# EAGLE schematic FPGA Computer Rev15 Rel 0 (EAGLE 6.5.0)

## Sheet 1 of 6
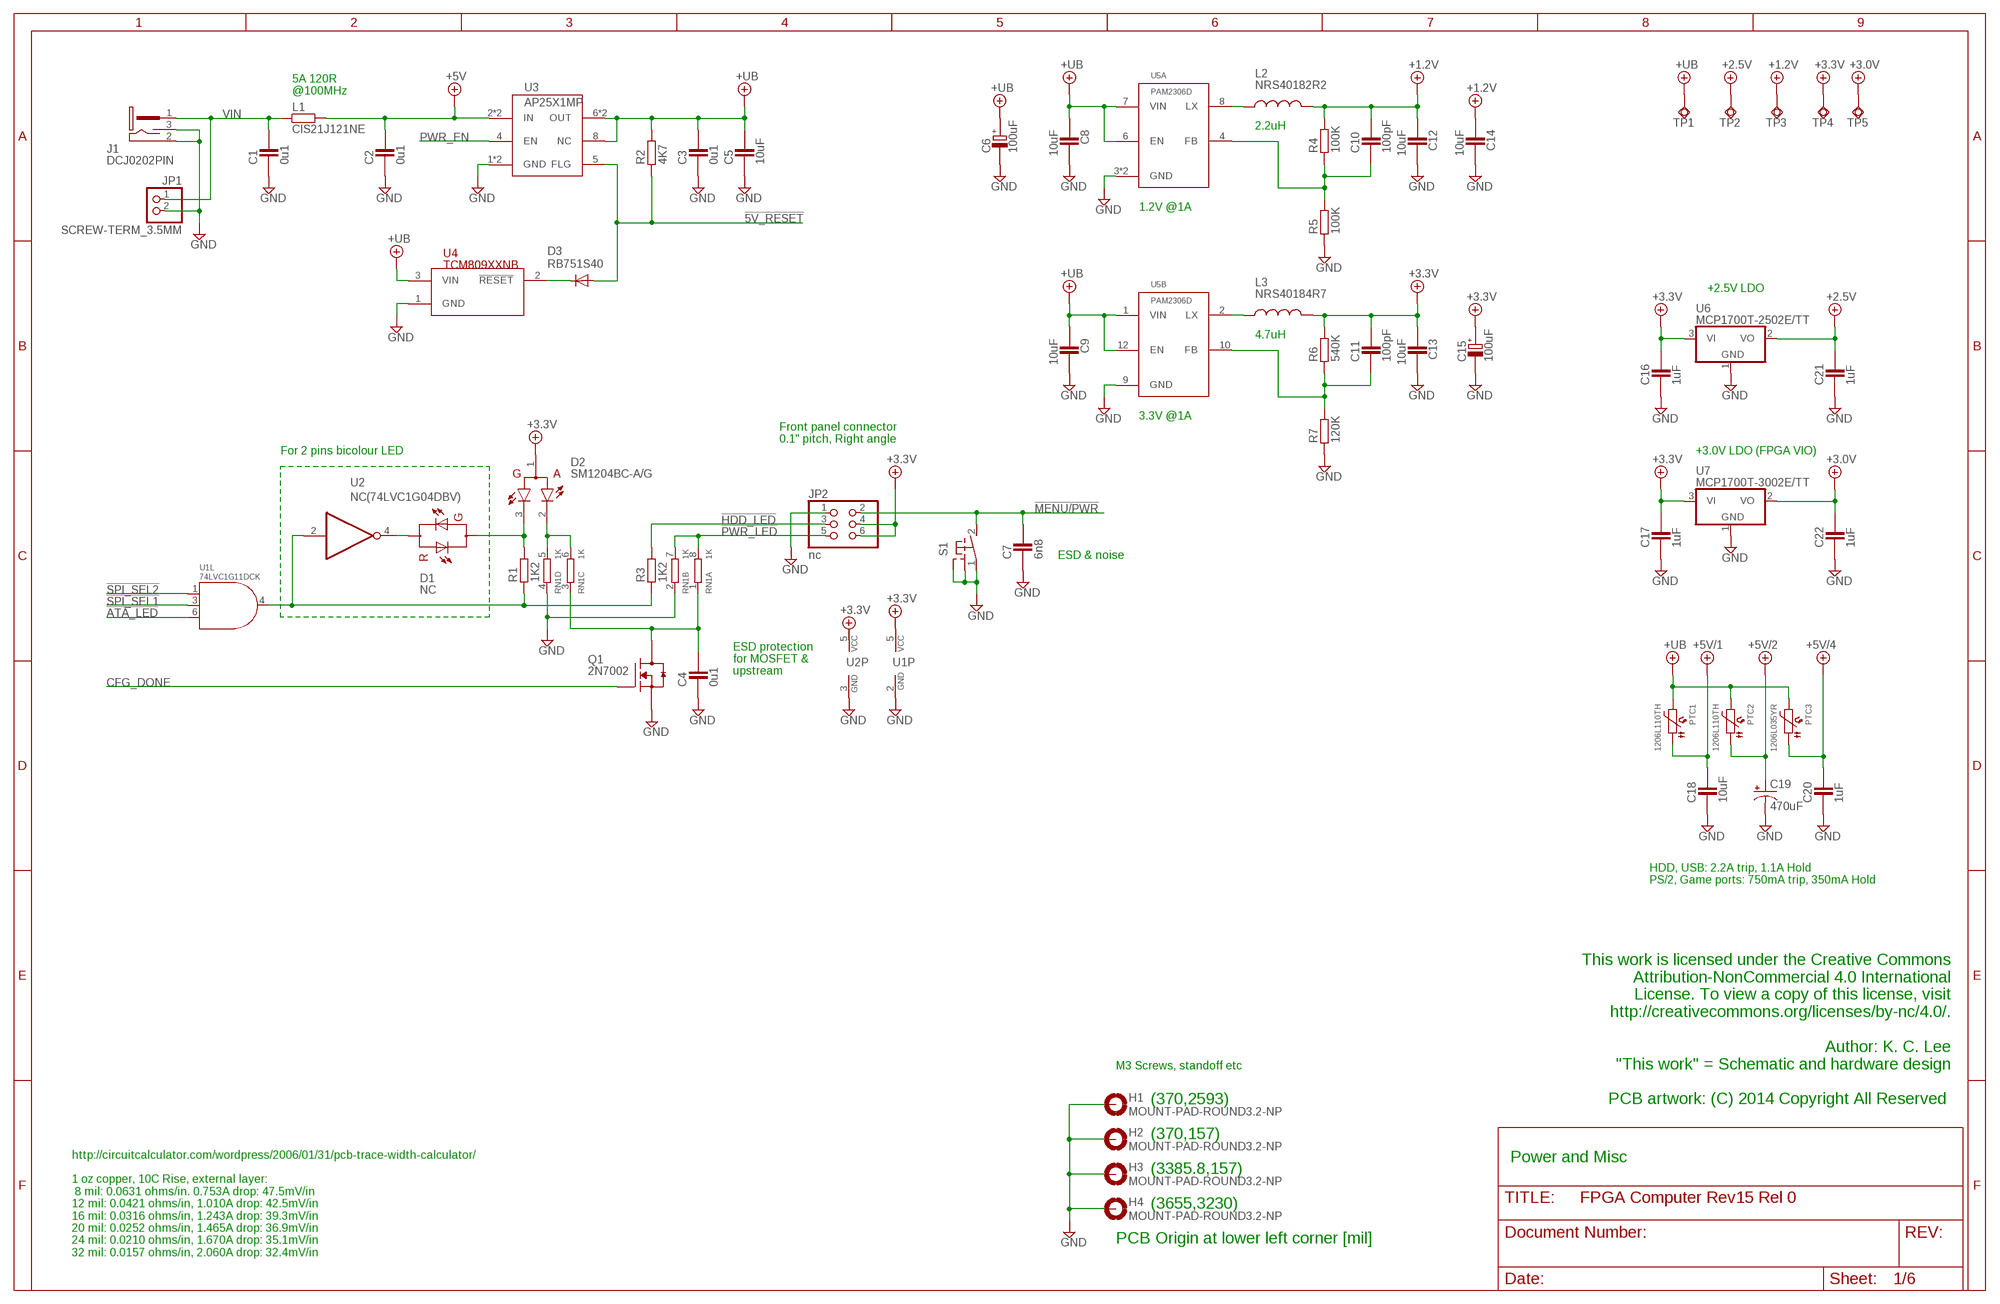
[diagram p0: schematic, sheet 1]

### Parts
C1  0u1  CAPACITOR_0603  [CAPC1608X92N]
C2  0u1  CAPACITOR_0603  [CAPC1608X92N]
C3  0u1  CAPACITOR_0603  [CAPC1608X92N]
C4  0u1  CAPACITOR_0603  [CAPC1608X92N]
C5  10uF  CAPACITOR_0805N  [CAP2012X70N]
C6  100uF  POLARISED_D_CASE  [CAPMP7343X310N]
C7  6n8  CAPACITOR_0603  [CAPC1608X92N]
C8  10uF  CAPACITOR_0805N  [CAP2012X70N]
C9  10uF  CAPACITOR_0805N  [CAP2012X70N]
C10  100pF  CAPACITOR_0603  [CAPC1608X92N]
C11  100pF  CAPACITOR_0603  [CAPC1608X92N]
C12  10uF  CAPACITOR_0805N  [CAP2012X70N]
C13  10uF  CAPACITOR_0805N  [CAP2012X70N]
C14  10uF  CAPACITOR_0805N  [CAP2012X70N]
C15  100uF  POLARISED_D_CASE  [CAPMP7343X310N]
C16  1uF  CAPACITOR_0603  [CAPC1608X92N]
C17  1uF  CAPACITOR_0603  [CAPC1608X92N]
C18  10uF  CAPACITOR_0805N  [CAP2012X70N]
C19  470uF  CAP_POL  [E2,5-6E]
C20  1uF  CAPACITOR_0603  [CAPC1608X92N]
C21  1uF  CAPACITOR_0603  [CAPC1608X92N]
C22  1uF  CAPACITOR_0603  [CAPC1608X92N]
D1  NC  DUAL-LED3MM  [LED3MM]
D2  SM1204BC-A/G  1204-SIDE-DUAL-AG  [LED_1204]
D3  RB751S40  DIODE-SOD523  [SOD523]
H1  MOUNT-PAD-ROUND3.2-NP  [3.2-PAD-NP]
H2  MOUNT-PAD-ROUND3.2-NP  [3.2-PAD-NP]
H3  MOUNT-PAD-ROUND3.2-NP  [3.2-PAD-NP]
H4  MOUNT-PAD-ROUND3.2-NP  [3.2-PAD-NP]
J1  DCJ0202PIN  [PJ-102A]
JP1  SCREW-TERM_3.5MM  [SCREWTERMINAL-3.5MM-2]
JP2  nc  PINHD-2X3_2.54-90°  [2X03-90]
L1  CIS21J121NE  RESISTOR_0805  [RESC2012X70N]
L2  NRS40182R2  NRS4018  [NR4018]
L3  NRS40184R7  NRS4018  [NR4018]
PTC1  1206L110TH  PTC1206  [1206]
PTC2  1206L110TH  PTC1206  [1206]
PTC3  1206L035YR  PTC1206  [1206]
Q1  2N7002  MOSFET-NCH_SOT-23  [SOT95P280X135-3N]
R1  1K2  RESISTOR_0603  [RESC1608X55N]
R2  4K7  RESISTOR_0603  [RESC1608X55N]
R3  1K2  RESISTOR_0603  [RESC1608X55N]
R4  100K  RESISTOR_0603  [RESC1608X55N]
R5  100K  RESISTOR_0603  [RESC1608X55N]
R6  540K  RESISTOR_0603  [RESC1608X55N]
R7  120K  RESISTOR_0603  [RESC1608X55N]
RN1  1K  4R-NCAT16  [CAT16]
S1  MOM_SW-RTPTS635V  [PTS635V]
TP1  TPSQTP07R  [TP07R]
TP2  TPSQTP07R  [TP07R]
TP3  TPSQTP07R  [TP07R]
TP4  TPSQTP07R  [TP07R]
TP5  TPSQTP07R  [TP07R]
U1  74LVC1G11DCK  [SC70-6]
U2  NC(74LVC1G04DBV)  74LVC1G04DBV  [SOT23-5]
U3  AP25X1MP  [MSOP8-PAD]
U4  TCM809XXNB  [SOT95P280X135-3N]
U5  PAM2306D  [PAM2306D]
U6  MCP1700T-2502E/TT  MCP1700/TT  [SOT95P280X135-3N]
U7  MCP1700T-3002E/TT  MCP1700/TT  [SOT95P280X135-3N]

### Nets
!5V_RESET: D3.A R2.1 U3.5(FLG) ; also sheet 3
!5V_RESET1: R1.1 R3.1 U1.4(L:Y) U2.2(I)
!ATA_LED: U1.6(L:C) ; also sheet 3
!HDD_LED: JP2.3 R3.2
!MENU/PWR: C7.2 JP2.2 S1.2(S) ; also sheet 4
!PWR_LED: JP2.5 RN1.7 RN1.8
!SPI_SEL1: U1.3(L:B) ; also sheet 2,4
!SPI_SEL2: U1.1(L:A) ; also sheet 2,4
+1.2V: C10.2 C12.1 C14.1 L2.2 R4.2 TP3.TP ; also sheet 5,6
+2.5V: C21.2 TP2.TP U6.2(VO) ; also sheet 5,6
+3.0V: C22.2 TP5.TP U7.2(VO) ; also sheet 5,6
+3.3V: C11.2 C13.1 C15.+ C16.2 C17.2 D2.1(A) JP2.4 JP2.6 L3.2 R6.2 TP4.TP U1.5(P:VCC) U2.5(VCC) U6.3(VI) U7.3(VI) ; also sheet 2,3,5
+5V: C2.2 L1.2 U3.2(IN) U3.3(IN) ; also sheet 4
+5V/1: C18.2 PTC1.1 ; also sheet 3
+5V/2: C19.+ PTC2.1 ; also sheet 4
+5V/4: C20.2 PTC3.1 ; also sheet 2
+UB: C3.2 C5.2 C6.+ C8.1 C9.1 PTC1.2 PTC2.2 PTC3.2 R2.2 TP1.TP U3.6(OUT) U3.7(OUT) U3.8(NC) U4.3(VIN) U5.1(B:VIN) U5.6(A:EN) U5.7(A:VIN) U5.12(B:EN) ; also sheet 2,5,6
CFG_DONE: Q1.1(G) ; also sheet 4,5
GND: C1.1 C2.1 C3.1 C4.1 C5.1 C6.- C7.1 C8.2 C9.2 C12.2 C13.2 C14.2 C15.- C16.1 C17.1 C18.1 C19.- C20.1 C21.1 C22.1 H1.H@1(MOUNT) H1.H@2(MOUNT) H1.H@3(MOUNT) H1.H@4(MOUNT) H1.H@5(MOUNT) H1.H@6(MOUNT) H1.H@7(MOUNT) H1.H@8(MOUNT) H2.H@1(MOUNT) H2.H@2(MOUNT) H2.H@3(MOUNT) H2.H@4(MOUNT) H2.H@5(MOUNT) H2.H@6(MOUNT) H2.H@7(MOUNT) H2.H@8(MOUNT) H3.H@1(MOUNT) H3.H@2(MOUNT) H3.H@3(MOUNT) H3.H@4(MOUNT) H3.H@5(MOUNT) H3.H@6(MOUNT) H3.H@7(MOUNT) H3.H@8(MOUNT) H4.H@1(MOUNT) H4.H@2(MOUNT) H4.H@3(MOUNT) H4.H@4(MOUNT) H4.H@5(MOUNT) H4.H@6(MOUNT) H4.H@7(MOUNT) H4.H@8(MOUNT) J1.2 J1.3 JP1.2 JP2.1 Q1.2(S) R5.1 R7.1 RN1.2 RN1.4 S1.1(P) S1.3(SHD) S1.4(SHD) U1.2(P:GND) U2.3(GND) U3.1(GND) U3.PAD(GND) U4.1(GND) U5.3(A:GND) U5.9(B:GND) U5.PAD(A:GND) U6.1(GND) U7.1(GND) ; also sheet 2,3,4,5,6
N$5: D3.C U4.2(!RESET)
N$25: D2.2(C2) RN1.5 RN1.6
N$60: C4.2 Q1.3(D) RN1.1 RN1.3
N$65: D1.A D2.3(C1) R1.2
N$84: C10.1 R4.1 R5.2 U5.4(A:FB)
N$85: L2.1 U5.8(A:LX)
N$87: C11.1 R6.1 R7.2 U5.10(B:FB)
N$88: L3.1 U5.2(B:LX)
N$98: D1.K(C) U2.4(O)
PWR_EN: U3.4(EN) ; also sheet 4
VIN: C1.2 J1.1 JP1.1 L1.1

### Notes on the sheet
- 5A 120R
  @100MHz
- 2.2uH
- 1.2V @1A
- +2.5V LDO
- 4.7uH
- 3.3V @1A
- Front panel connector
  0.1" pitch, Right angle
- For 2 pins bicolour LED | +3.0V LDO (FPGA VIO)
- ESD & noise
- ESD protection
  for MOSFET &
  upstream
- HDD, USB: 2.2A trip, 1.1A Hold
  PS/2, Game ports: 750mA trip, 350mA Hold
- M3 Screws, standoff etc
- (370,2593)
- This work is licensed under the Creative Commons
  Attribution-NonCommercial 4.0 International
  License. To view a copy of this license, visit
  http://creativecommons.org/licenses/by-nc/4.0/.
  
  Author: K. C. Lee
  "This work" = Schematic and hardware design
  
  PCB artwork: (C) 2014 Copyright All Reserved
- (370,157)
- http://circuitcalculator.com/wordpress/2006/01/31/pcb-trace-width-calculator/
  
  1 oz copper, 10C Rise, external layer:
   8 mil: 0.0631 ohms/in. 0.753A drop: 47.5mV/in
  12 mil: 0.0421 ohms/in, 1.010A drop: 42.5mV/in
  16 mil: 0.0316 ohms/in, 1.243A drop: 39.3mV/in
  20 mil: 0.0252 ohms/in, 1.465A drop: 36.9mV/in
  24 mil: 0.0210 ohms/in, 1.670A drop: 35.1mV/in
  32 mil: 0.0157 ohms/in, 2.060A drop: 32.4mV/in
- Power and Misc
- (3385.8,157)
- (3655,3230)
- PCB Origin at lower left corner [mil]

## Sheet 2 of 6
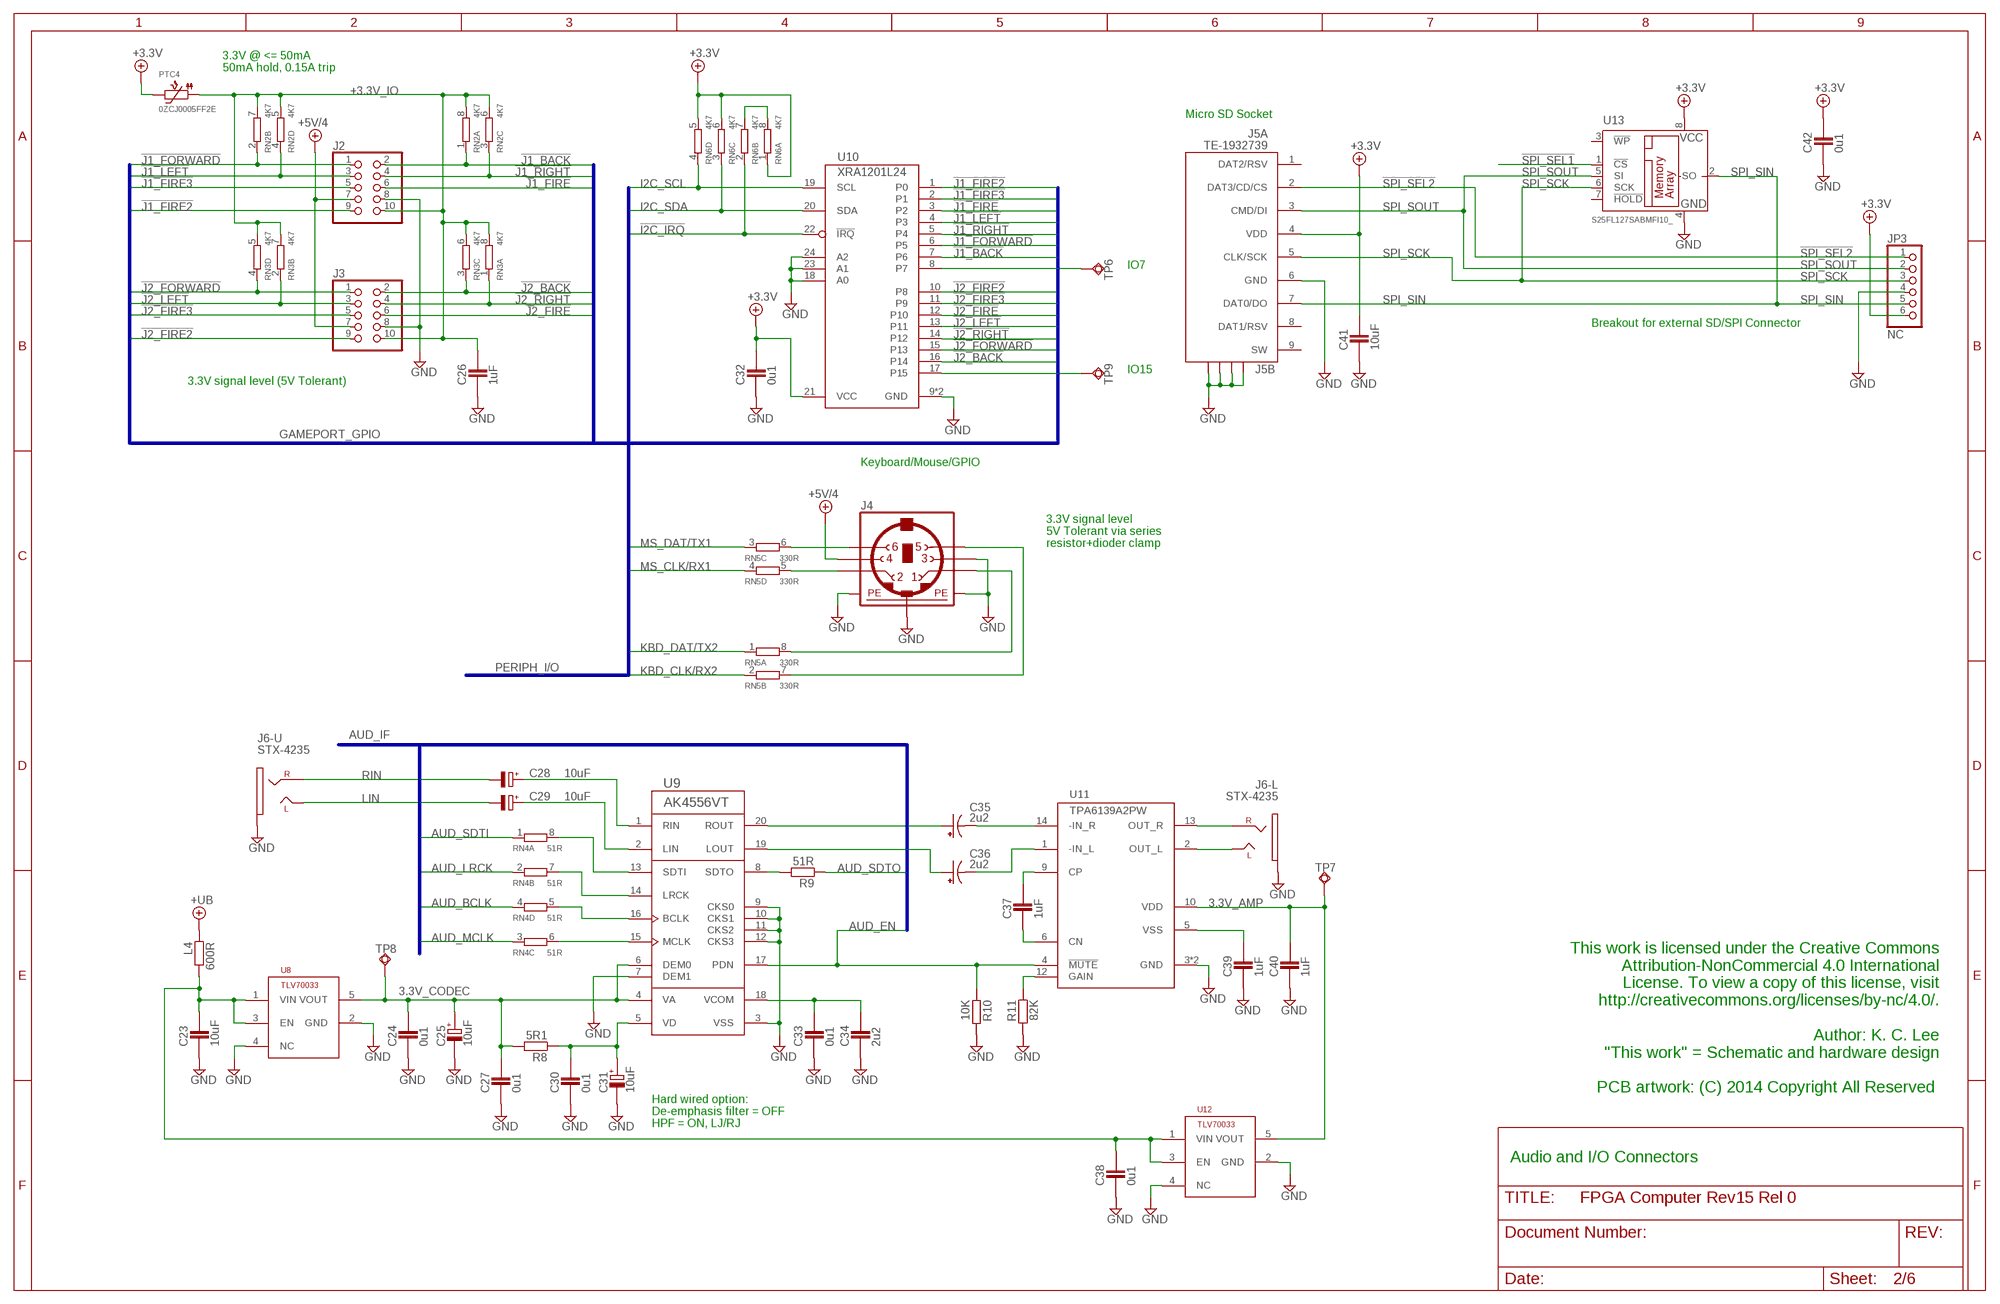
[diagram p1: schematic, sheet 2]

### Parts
C23  10uF  CAPACITOR_0805N  [CAP2012X70N]
C24  0u1  CAPACITOR_0603  [CAPC1608X92N]
C25  10uF  POLARISED_B_CASE  [CAPMP3528X210N]
C26  1uF  CAPACITOR_0603  [CAPC1608X92N]
C27  0u1  CAPACITOR_0603  [CAPC1608X92N]
C28  10uF  CPOL-EUE2-5  [E2-5]
C29  10uF  CPOL-EUE2-5  [E2-5]
C30  0u1  CAPACITOR_0603  [CAPC1608X92N]
C31  10uF  POLARISED_B_CASE  [CAPMP3528X210N]
C32  0u1  CAPACITOR_0603  [CAPC1608X92N]
C33  0u1  CAPACITOR_0603  [CAPC1608X92N]
C34  2u2  CAPACITOR_0603  [CAPC1608X92N]
C35  2u2  C-PR-1,0X3  [E1,0-3]
C36  2u2  C-PR-1,0X3  [E1,0-3]
C37  1uF  CAPACITOR_0603  [CAPC1608X92N]
C38  0u1  CAPACITOR_0603  [CAPC1608X92N]
C39  1uF  CAPACITOR_0603  [CAPC1608X92N]
C40  1uF  CAPACITOR_0603  [CAPC1608X92N]
C41  10uF  CAPACITOR_0805N  [CAP2012X70N]
C42  0u1  CAPACITOR_0603  [CAPC1608X92N]
J2  PINHD-2X5_2.54-W/PLUG  [2X05-W_PLUG]
J3  PINHD-2X5_2.54-W/PLUG  [2X05-W_PLUG]
J4  MINI_DIN_6  [M_DIN6]
J5  TE-1932739  [TE-1932739]
J6  STX-4235  [STX-4235-3]
JP3  NC  PINHD-1X6_2.00  [1X06M]
L4  600R  RESISTOR_0603  [RESC1608X55N]
PTC4  0ZCJ0005FF2E  PTC1206  [1206]
R8  5R1  RESISTOR_0603  [RESC1608X55N]
R9  51R  RESISTOR_0603  [RESC1608X55N]
R10  10K  RESISTOR_0603  [RESC1608X55N]
R11  82K  RESISTOR_0603  [RESC1608X55N]
RN2  4K7  4R-NCAT16  [CAT16]
RN3  4K7  4R-NCAT16  [CAT16]
RN4  51R  4R-NCAT16  [CAT16]
RN5  330R  4R-NCAT16  [CAT16]
RN6  4K7  4R-NCAT16  [CAT16]
TP6  TPSQTP07R  [TP07R]
TP7  TPSQTP07R  [TP07R]
TP8  TPSQTP07R  [TP07R]
TP9  TPSQTP07R  [TP07R]
U8  TLV70033  LDO-5  [SOT23-5]
U9  AK4556VT  [TSSOP20]
U10  XRA1201L24  [S-PQFP-N24-PAD]
U11  TPA6139A2PW  [TSSOP14]
U12  TLV70033  LDO-5  [SOT23-5]
U13  S25FL127SABMFI10_  25LC080SN  [SO-08]

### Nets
3.3V_AMP: C40.2 TP7.TP U11.10(VDD) U12.5(VOUT)
3.3V_CODEC: C24.2 C25.+ C27.2 R8.2 TP8.TP U8.5(VOUT) U9.4(VA) U9.6(DEM0)
!I2C_IRQ: RN6.2 U10.22(!IRQ) ; also sheet 4,6
!J1_BACK: J2.2 RN2.1 U10.7(P6)
!J1_FIRE: J2.6 U10.3(P2)
!J1_FIRE2: J2.9 U10.1(P0)
!J1_FIRE3: J2.5 U10.2(P1)
!J1_FORWARD: J2.1 RN2.2 U10.6(P5)
!J1_LEFT: J2.3 RN2.4 U10.4(P3)
!J1_RIGHT: J2.4 RN2.3 U10.5(P4)
!J2_BACK: J3.2 RN3.3 U10.16(P14)
!J2_FIRE: J3.6 U10.12(P10)
!J2_FIRE2: J3.9 U10.10(P8)
!J2_FIRE3: J3.5 U10.11(P9)
!J2_FORWARD: J3.1 RN3.4 U10.15(P13)
!J2_LEFT: J3.3 RN3.2 U10.13(P11)
!J2_RIGHT: J3.4 RN3.1 U10.14(P12)
!SPI_SEL1: U13.1(!CS) ; also sheet 1,4
!SPI_SEL2: J5.2(A:DAT3/CD/CS) JP3.1 ; also sheet 1,4
+3.3V: C32.2 C41.2 C42.2 J5.4(A:VDD) JP3.6 PTC4.2 RN6.1 RN6.5 RN6.6 U10.21(VCC) U13.8(VCC) ; also sheet 1,3,5
+3.3V_IO: C26.2 J2.10 J3.10 PTC4.1 RN2.5 RN2.6 RN2.7 RN2.8 RN3.5 RN3.6 RN3.7 RN3.8
+5V/4: J2.7 J3.7 J4.4 ; also sheet 1
+UB: L4.1 ; also sheet 1,5,6
AUD_BCLK: RN4.4 ; also sheet 5
AUD_EN: R10.1 U9.17(PDN) U11.4(!MUTE) ; also sheet 6
AUD_LRCK: RN4.2 ; also sheet 5
AUD_MCLK: RN4.3 ; also sheet 5
AUD_SDTI: RN4.1 ; also sheet 5
AUD_SDTO: R9.1 ; also sheet 5
GND: C23.1 C24.1 C25.- C26.1 C27.1 C30.1 C31.- C32.1 C33.1 C34.1 C38.1 C39.1 C40.1 C41.1 C42.1 J2.8 J3.8 J4.3 J4.SH1(PE1) J4.SH2(PE2) J4.SH3(PE3) J5.6(A:GND) J5.G1(B:S1) J5.G2(B:S2) J5.G3(B:S3) J5.G4(B:S4) J6.5L J6.5U JP3.4 R10.2 R11.2 U8.2(GND) U8.4(NC) U9.3(VSS) U9.7(DEM1) U9.9(CKS0) U9.10(CKS1) U9.11(CKS2) U9.12(CKS3) U10.9(GND) U10.18(A0) U10.23(A1) U10.24(A2) U10.PAD(GND) U11.3(GND) U11.11(GND) U12.2(GND) U12.4(NC) U13.4(GND) ; also sheet 1,3,4,5,6
I2C_SCL: RN6.4 U10.19(SCL) ; also sheet 4,6
I2C_SDA: RN6.3 U10.20(SDA) ; also sheet 4,6
KBD_CLK/RX2: RN5.2 ; also sheet 4
KBD_DAT/TX2: RN5.1 ; also sheet 4
LIN: C29.- J6.4U
MS_CLK/RX1: RN5.4 ; also sheet 4
MS_DAT/TX1: RN5.3 ; also sheet 4
N$1: J4.6 RN5.6
N$9: C23.2 C38.2 L4.2 U8.1(VIN) U8.3(EN) U12.1(VIN) U12.3(EN)
N$12: C36.- U11.1(-IN_L)
N$15: RN6.7 RN6.8
N$17: J4.1 RN5.8
N$19: J4.5 RN5.7
N$20: R11.1 U11.12(GAIN)
N$22: C37.1 U11.6(CN)
N$24: C37.2 U11.9(CP)
N$29: J6.4L U11.2(OUT_L)
N$30: J6.1L U11.13(OUT_R)
N$31: C39.2 U11.5(VSS)
N$51: J4.2 RN5.5
N$54: C35.- U11.14(-IN_R)
N$61: TP9.TP U10.17(P15)
N$66: C29.+ U9.2(LIN)
N$67: C28.+ U9.1(RIN)
N$69: R9.2 U9.8(SDTO)
N$70: C30.2 C31.+ R8.1 U9.5(VD)
N$71: RN4.6 U9.15(MCLK)
N$72: RN4.5 U9.16(BCLK)
N$75: RN4.7 U9.14(LRCK)
N$76: RN4.8 U9.13(SDTI)
N$80: C33.2 C34.2 U9.18(VCOM)
N$81: C35.+ U9.20(ROUT)
N$82: C36.+ U9.19(LOUT)
N$93: TP6.TP U10.8(P7)
RIN: C28.- J6.1U
SPI_SCK: J5.5(A:CLK/SCK) JP3.3 U13.6(SCK) ; also sheet 3,4,6
SPI_SIN: J5.7(A:DAT0/DO) JP3.5 U13.2(SO) ; also sheet 3,4
SPI_SOUT: J5.3(A:CMD/DI) JP3.2 U13.5(SI) ; also sheet 3,4,6
Unconnected: J5.1(A:DAT2/RSV) J5.8(A:DAT1/RSV) J5.9(A:SW) U13.3(!WP) U13.7(!HOLD)

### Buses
GAMEPORT_GPIO
AUD_IF
PERIPH_I/O

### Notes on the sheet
- 3.3V @ <= 50mA
  50mA hold, 0.15A trip
- Micro SD Socket
- IO7
- Breakout for external SD/SPI Connector
- IO15
- 3.3V signal level (5V Tolerant)
- Keyboard/Mouse/GPIO
- 3.3V signal level
  5V Tolerant via series 
  resistor+dioder clamp
- This work is licensed under the Creative Commons
  Attribution-NonCommercial 4.0 International
  License. To view a copy of this license, visit
  http://creativecommons.org/licenses/by-nc/4.0/.
  
  Author: K. C. Lee
  "This work" = Schematic and hardware design
  
  PCB artwork: (C) 2014 Copyright All Reserved
- Hard wired option:
  De-emphasis filter = OFF
  HPF = ON, LJ/RJ
- Audio and I/O Connectors

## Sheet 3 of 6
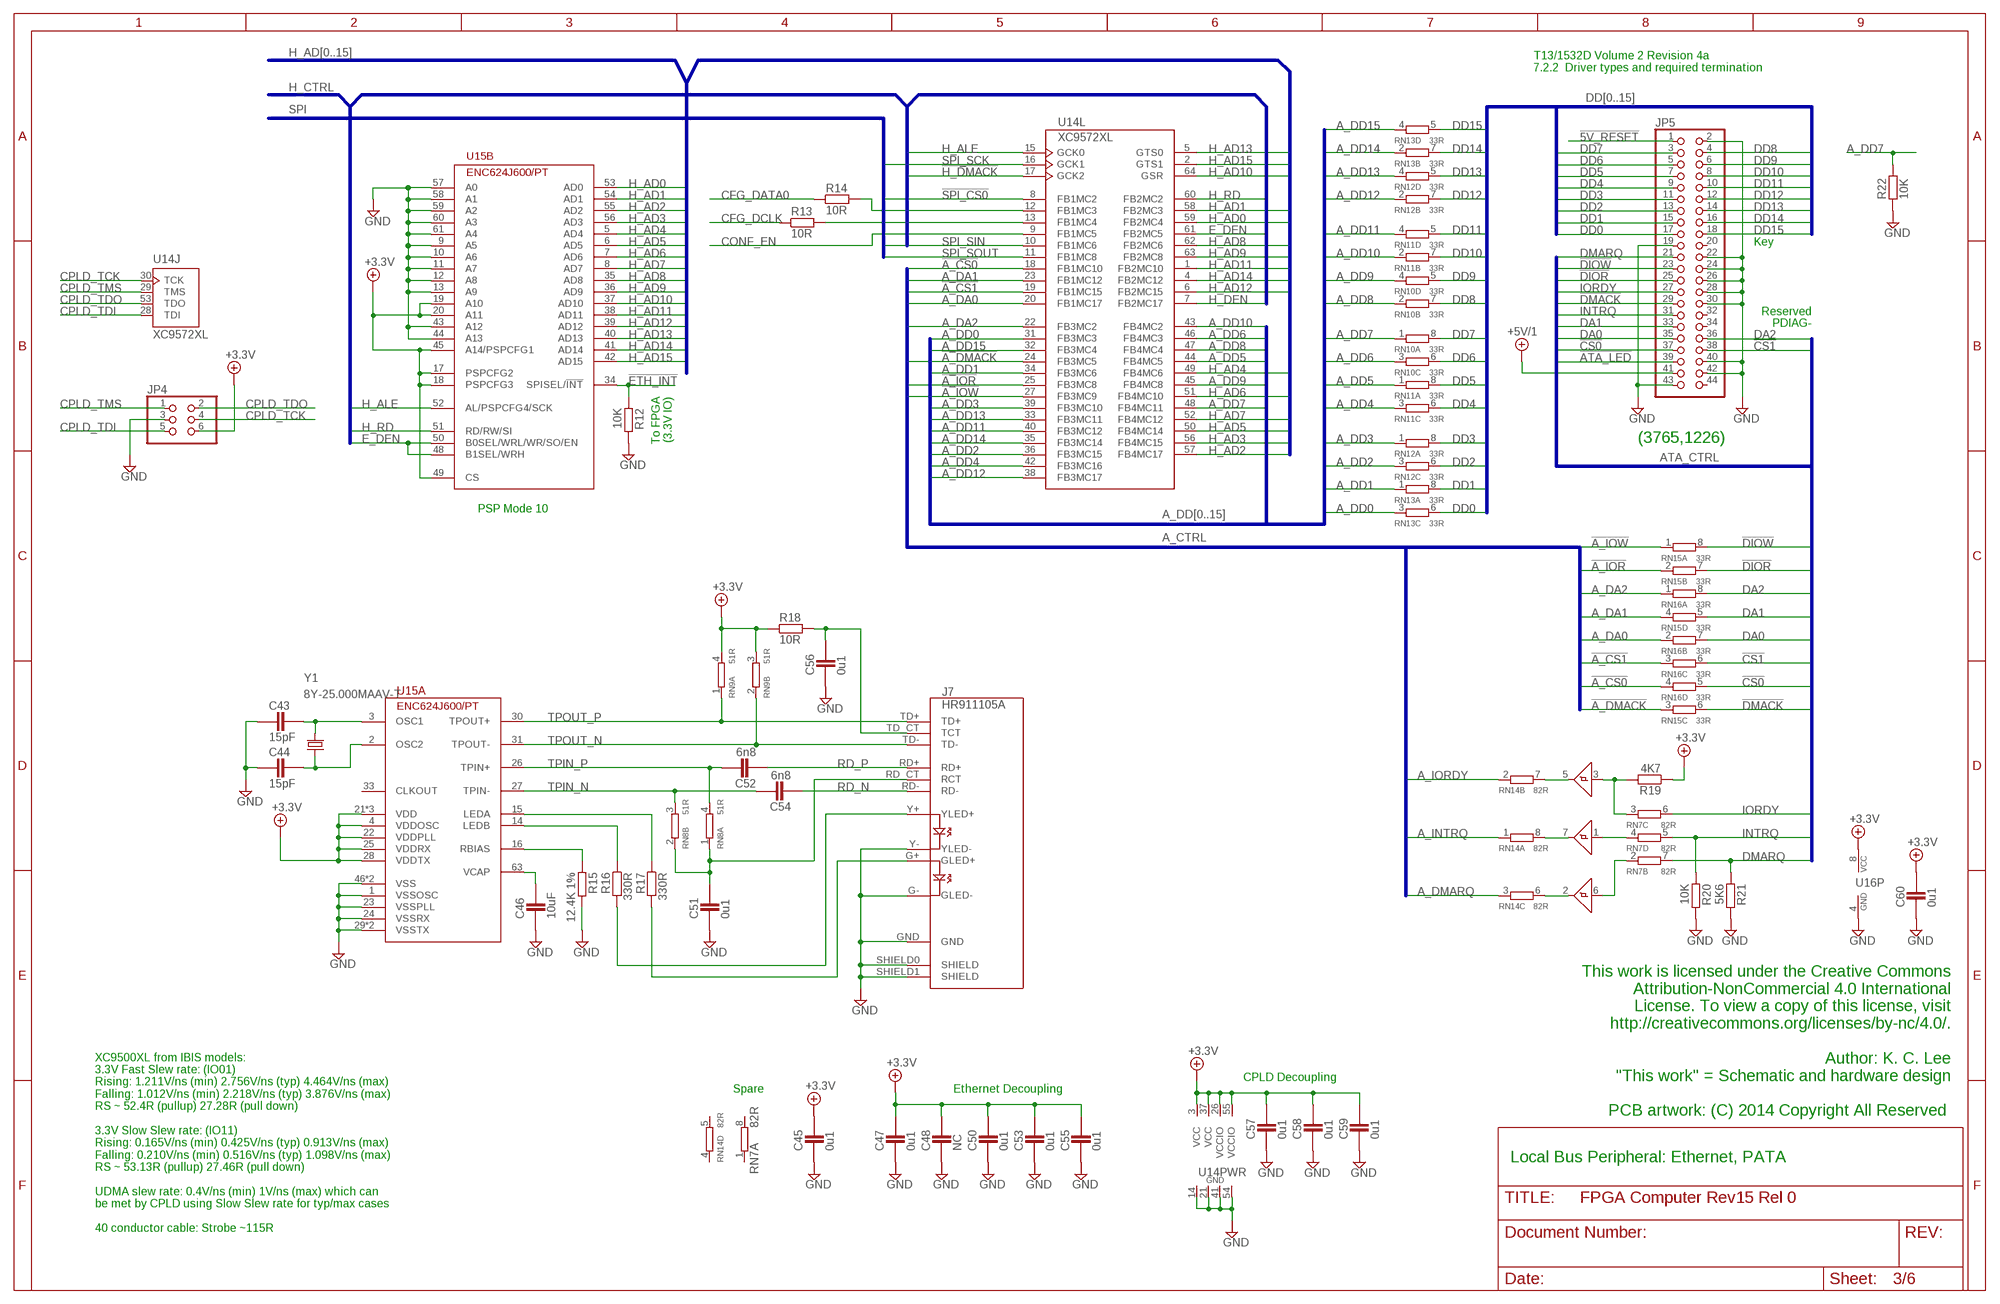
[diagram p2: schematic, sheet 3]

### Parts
C43  15pF  CAPACITOR_0603  [CAPC1608X92N]
C44  15pF  CAPACITOR_0603  [CAPC1608X92N]
C45  0u1  CAPACITOR_0603  [CAPC1608X92N]
C46  10uF  CAPACITOR_0805N  [CAP2012X70N]
C47  0u1  CAPACITOR_0603  [CAPC1608X92N]
C48  NC  CAPACITOR_0603  [CAPC1608X92N]
C50  0u1  CAPACITOR_0603  [CAPC1608X92N]
C51  0u1  CAPACITOR_0402  [CAPC1005X60N]
C52  6n8  CAPACITOR_0603  [CAPC1608X92N]
C53  0u1  CAPACITOR_0402  [CAPC1005X60N]
C54  6n8  CAPACITOR_0603  [CAPC1608X92N]
C55  0u1  CAPACITOR_0603  [CAPC1608X92N]
C56  0u1  CAPACITOR_0402  [CAPC1005X60N]
C57  0u1  CAPACITOR_0402  [CAPC1005X60N]
C58  0u1  CAPACITOR_0402  [CAPC1005X60N]
C59  0u1  CAPACITOR_0402  [CAPC1005X60N]
C60  0u1  CAPACITOR_0603  [CAPC1608X92N]
J7  HR911105A  [HR911105A]
JP4  PINHD-2X3_2.54-ROUND  [2X03-RND]
JP5  PINHD-2X22_2.00-W/PLUG  [2X22M-W_PLUG]
R12  10K  RESISTOR_0603  [RESC1608X55N]
R13  10R  RESISTOR_0603  [RESC1608X55N]
R14  10R  RESISTOR_0603  [RESC1608X55N]
R15  12.4K 1%  RESISTOR_0603  [RESC1608X55N]
R16  330R  RESISTOR_0603  [RESC1608X55N]
R17  330R  RESISTOR_0603  [RESC1608X55N]
R18  10R  RESISTOR_0603  [RESC1608X55N]
R19  4K7  RESISTOR_0603  [RESC1608X55N]
R20  10K  RESISTOR_0603  [RESC1608X55N]
R21  5K6  RESISTOR_0603  [RESC1608X55N]
R22  10K  RESISTOR_0603  [RESC1608X55N]
RN7  82R  4R-NCAT16  [CAT16]
RN8  51R  2R-NEXBV4V  [EXBV4V]
RN9  51R  2R-NEXBV4V  [EXBV4V]
RN10  33R  4R-NCAT16  [CAT16]
RN11  33R  4R-NCAT16  [CAT16]
RN12  33R  4R-NCAT16  [CAT16]
RN13  33R  4R-NCAT16  [CAT16]
RN14  82R  4R-NCAT16  [CAT16]
RN15  33R  4R-NCAT16  [CAT16]
RN16  33R  4R-NCAT16  [CAT16]
U14  XC9572XL  XC9572VQ64  [TQFP64]
U15  ENC624J600/PT  [TQFP64]
U16  74LVC3G17DCU  [MAB08A]
Y1  8Y-25.000MAAV-T  XTAL_XRCGB  [XTAL_2.0X1.6]

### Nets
!5V_RESET: JP5.1 ; also sheet 1
!A_CS0: RN16.4 U14.18(L:FB1MC10)
!A_CS1: RN16.3 U14.19(L:FB1MC15)
!A_DMACK: RN15.3 U14.24(L:FB3MC5)
!A_IOR: RN15.2 U14.25(L:FB3MC8)
!A_IOW: RN15.1 U14.27(L:FB3MC9)
!ATA_LED: JP5.39 ; also sheet 1
!CS0: JP5.37 RN16.5
!CS1: JP5.38 RN16.6
!DIOR: JP5.25 RN15.7
!DIOW: JP5.23 RN15.8
!DMACK: JP5.29 RN15.6
!ETH_INT: R12.1 U15.34(B:SPISEL/!INT!) ; also sheet 4,6
!H_DMACK: U14.17(L:GCK2) ; also sheet 6
!SPI_CS0: U14.8(L:FB1MC2) ; also sheet 4,6
+3.3V: C45.2 C47.2 C48.2 C50.2 C53.2 C55.2 C57.2 C58.2 C59.2 C60.2 JP4.6 R18.1 R19.1 RN9.3 RN9.4 U14.3(PWR:VCC) U14.26(PWR:VCCIO) U14.37(PWR:VCC) U14.55(PWR:VCCIO) U15.4(A:VDDOSC) U15.17(B:PSPCFG2) U15.18(B:PSPCFG3) U15.19(B:A10) U15.20(B:A11) U15.21(A:VDD) U15.22(A:VDDPLL) U15.25(A:VDDRX) U15.28(A:VDDTX) U15.45(B:A14/PSPCFG1) U15.47(A:VDD) U15.49(B:CS) U15.64(A:VDD) U16.8(P:VCC) ; also sheet 1,2,5
+5V/1: JP5.41 ; also sheet 1
A_DA0: RN16.2 U14.20(L:FB1MC17)
A_DA1: RN15.4 U14.23(L:FB1MC12)
A_DA2: RN16.1 U14.22(L:FB3MC2)
A_DD0: RN13.3 U14.31(L:FB3MC3)
A_DD1: RN13.1 U14.34(L:FB3MC6)
A_DD2: RN12.3 U14.36(L:FB3MC15)
A_DD3: RN12.1 U14.39(L:FB3MC10)
A_DD4: RN11.3 U14.42(L:FB3MC16)
A_DD5: RN11.1 U14.44(L:FB4MC5)
A_DD6: RN10.3 U14.46(L:FB4MC3)
A_DD7: R22.2 RN10.1 U14.48(L:FB4MC11)
A_DD8: RN10.2 U14.47(L:FB4MC4)
A_DD9: RN10.4 U14.45(L:FB4MC8)
A_DD10: RN11.2 U14.43(L:FB4MC2)
A_DD11: RN11.4 U14.40(L:FB3MC12)
A_DD12: RN12.2 U14.38(L:FB3MC17)
A_DD13: RN12.4 U14.33(L:FB3MC11)
A_DD14: RN13.2 U14.35(L:FB3MC14)
A_DD15: RN13.4 U14.32(L:FB3MC4)
A_DMARQ: RN14.3 ; also sheet 6
A_INTRQ: RN14.1 ; also sheet 6
A_IORDY: RN14.2 ; also sheet 6
CFG_DATA0: R14.1 ; also sheet 5
CFG_DCLK: R13.1 ; also sheet 5
CONF_EN: U14.9(L:FB1MC5) ; also sheet 4
CPLD_TCK: JP4.4 U14.30(J:TCK)
CPLD_TDI: JP4.5 U14.28(J:TDI)
CPLD_TDO: JP4.2 U14.53(J:TDO)
CPLD_TMS: JP4.1 U14.29(J:TMS)
DA0: JP5.35 RN16.7
DA1: JP5.33 RN15.5
DA2: JP5.36 RN16.8
DD0: JP5.17 RN13.6
DD1: JP5.15 RN13.8
DD2: JP5.13 RN12.6
DD3: JP5.11 RN12.8
DD4: JP5.9 RN11.6
DD5: JP5.7 RN11.8
DD6: JP5.5 RN10.6
DD7: JP5.3 RN10.8
DD8: JP5.4 RN10.7
DD9: JP5.6 RN10.5
DD10: JP5.8 RN11.7
DD11: JP5.10 RN11.5
DD12: JP5.12 RN12.7
DD13: JP5.14 RN12.5
DD14: JP5.16 RN13.7
DD15: JP5.18 RN13.5
DMARQ: JP5.21 R21.1 RN7.7
E_DEN: U14.61(L:FB2MC5) U15.48(B:B1SEL/WRH) U15.50(B:B0SEL/WRL/WR/SO/EN)
GND: C43.1 C44.1 C45.1 C46.1 C47.1 C48.1 C50.1 C51.1 C53.1 C55.1 C56.1 C57.1 C58.1 C59.1 C60.1 J7.G-(GLED-) J7.GND J7.SHIELD0(SHIELD) J7.SHIELD1(SHIELD) J7.Y-(YLED-) JP4.3 JP5.2 JP5.19 JP5.22 JP5.24 JP5.26 JP5.28 JP5.30 JP5.40 JP5.42 JP5.43 R12.2 R15.2 R20.2 R21.2 R22.1 U14.14(PWR:GND) U14.21(PWR:GND) U14.41(PWR:GND) U14.54(PWR:GND) U15.1(A:VSSOSC) U15.9(B:A5) U15.10(B:A6) U15.11(B:A7) U15.12(B:A8) U15.13(B:A9) U15.23(A:VSSPLL) U15.24(A:VSSRX) U15.29(A:VSSTX) U15.32(A:VSSTX) U15.43(B:A12) U15.44(B:A13) U15.46(A:VSS) U15.57(B:A0) U15.58(B:A1) U15.59(B:A2) U15.60(B:A3) U15.61(B:A4) U15.62(A:VSS) U16.4(P:GND) ; also sheet 1,2,4,5,6
H_AD0: U14.59(L:FB2MC4) U15.53(B:AD0) ; also sheet 6
H_AD1: U14.58(L:FB2MC3) U15.54(B:AD1) ; also sheet 6
H_AD2: U14.57(L:FB4MC17) U15.55(B:AD2) ; also sheet 6
H_AD3: U14.56(L:FB4MC15) U15.56(B:AD3) ; also sheet 6
H_AD4: U14.49(L:FB4MC6) U15.5(B:AD4) ; also sheet 6
H_AD5: U14.50(L:FB4MC14) U15.6(B:AD5) ; also sheet 6
H_AD6: U14.51(L:FB4MC10) U15.7(B:AD6) ; also sheet 6
H_AD7: U14.52(L:FB4MC12) U15.8(B:AD7) ; also sheet 6
H_AD8: U14.62(L:FB2MC6) U15.35(B:AD8) ; also sheet 6
H_AD9: U14.63(L:FB2MC8) U15.36(B:AD9) ; also sheet 6
H_AD10: U14.64(L:GSR) U15.37(B:AD10) ; also sheet 6
H_AD11: U14.1(L:FB2MC10) U15.38(B:AD11) ; also sheet 6
H_AD12: U14.6(L:FB2MC15) U15.39(B:AD12) ; also sheet 6
H_AD13: U14.5(L:GTS0) U15.40(B:AD13) ; also sheet 6
H_AD14: U14.4(L:FB2MC12) U15.41(B:AD14) ; also sheet 6
H_AD15: U14.2(L:GTS1) U15.42(B:AD15) ; also sheet 6
H_ALE: U14.15(L:GCK0) U15.52(B:AL/PSPCFG4/SCK) ; also sheet 6
H_DEN: U14.7(L:FB2MC17) ; also sheet 6
H_RD: U14.60(L:FB2MC2) U15.51(B:RD/RW/SI) ; also sheet 6
INTRQ: JP5.31 R20.1 RN7.5
IORDY: JP5.27 RN7.6
N$3: C46.2 U15.63(A:VCAP)
N$4: C51.2 J7.RD_CT(RCT) RN8.1 RN8.2
N$10: R16.1 U15.14(A:LEDB)
N$11: J7.Y+(YLED+) R16.2
N$13: R17.1 U15.15(A:LEDA)
N$14: R15.1 U15.16(A:RBIAS)
N$16: C56.2 J7.TD_CT(TCT) R18.2
N$18: J7.G+(GLED+) R17.2
N$28: C43.2 U15.3(A:OSC1) Y1.3
N$32: RN14.7 U16.5(Y)
N$56: C44.2 U15.2(A:OSC2) Y1.1
N$83: RN14.8 U16.7(Y)
N$86: RN14.6 U16.2(Y)
N$90: R14.2 U14.12(L:FB1MC3)
N$91: R13.2 U14.13(L:FB1MC4)
N$106: RN7.2 U16.6(A)
N$107: RN7.4 U16.1(A)
N$109: R19.2 RN7.3 U16.3(A)
RD_N [diff2]: C54.1 J7.RD-
RD_P [diff2]: C52.1 J7.RD+
SPI_SCK: U14.16(L:GCK1) ; also sheet 2,4,6
SPI_SIN: U14.10(L:FB1MC6) ; also sheet 2,4
SPI_SOUT: U14.11(L:FB1MC8) ; also sheet 2,4,6
TPIN_N [diff2]: C54.2 RN8.3 U15.27(A:TPIN-)
TPIN_P [diff2]: C52.2 RN8.4 U15.26(A:TPIN+)
TPOUT_N [diff2]: J7.TD- RN9.2 U15.31(A:TPOUT-)
TPOUT_P [diff2]: J7.TD+ RN9.1 U15.30(A:TPOUT+)
Unconnected: JP5.20 JP5.32 JP5.34 JP5.44 RN7.1 RN7.8 RN14.4 RN14.5 U15.33(A:CLKOUT)

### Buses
DD[0..15]
A_DD[0..15]
H_CTRL
ATA_CTRL
A_CTRL
H_AD[0..15]
SPI

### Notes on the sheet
- T13/1532D Volume 2 Revision 4a 
  7.2.2  Driver types and required termination
- Key
- Reserved
- PDIAG-
- To FPGA
  (3.3V IO)
- (3765,1226)
- PSP Mode 10
- CPLD Decoupling
- Spare | Ethernet Decoupling
- This work is licensed under the Creative Commons
  Attribution-NonCommercial 4.0 International
  License. To view a copy of this license, visit
  http://creativecommons.org/licenses/by-nc/4.0/.
  
  Author: K. C. Lee
  "This work" = Schematic and hardware design
  
  PCB artwork: (C) 2014 Copyright All Reserved
- Local Bus Peripheral: Ethernet, PATA
- XC9500XL from IBIS models:
  3.3V Fast Slew rate: (IO01)
  Rising: 1.211V/ns (min) 2.756V/ns (typ) 4.464V/ns (max)
  Falling: 1.012V/ns (min) 2.218V/ns (typ) 3.876V/ns (max)
  RS ~ 52.4R (pullup) 27.28R (pull down)
  
  3.3V Slow Slew rate: (IO11)
  Rising: 0.165V/ns (min) 0.425V/ns (typ) 0.913V/ns (max)
  Falling: 0.210V/ns (min) 0.516V/ns (typ) 1.098V/ns (max)
  RS ~ 53.13R (pullup) 27.46R (pull down)
  
  UDMA slew rate: 0.4V/ns (min) 1V/ns (max) which can
  be met by CPLD using Slow Slew rate for typ/max cases
  
  40 conductor cable: Strobe ~115R

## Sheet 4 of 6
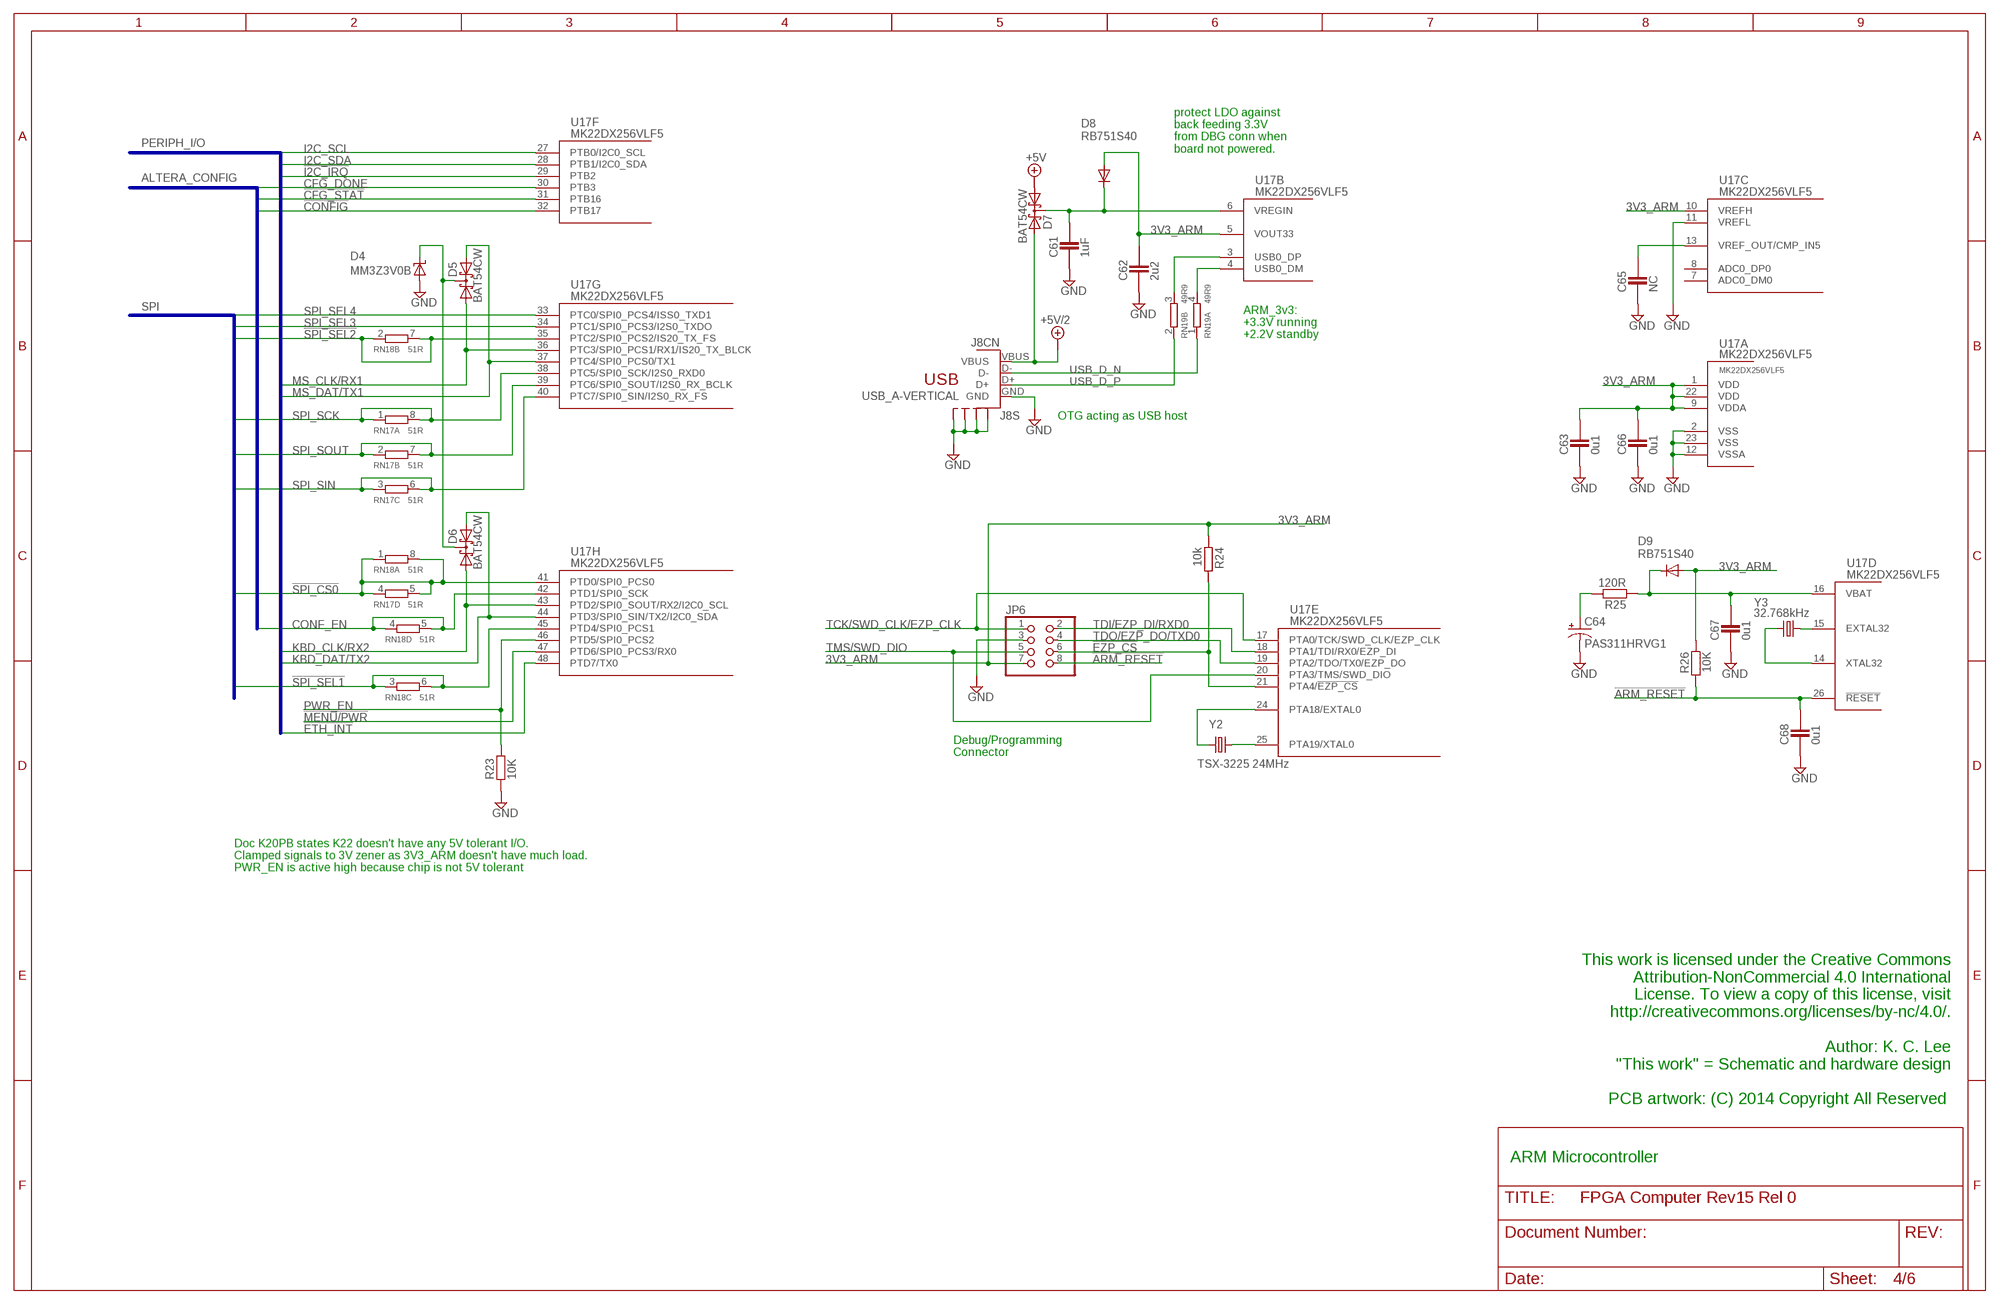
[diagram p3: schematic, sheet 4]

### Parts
C61  1uF  CAPACITOR_0603  [CAPC1608X92N]
C62  2u2  CAPACITOR_0603  [CAPC1608X92N]
C63  0u1  CAPACITOR_0603  [CAPC1608X92N]
C64  PAS311HRVG1  [311HR-VG1]
C65  NC  CAPACITOR_0603  [CAPC1608X92N]
C66  0u1  CAPACITOR_0603  [CAPC1608X92N]
C67  0u1  CAPACITOR_0603  [CAPC1608X92N]
C68  0u1  CAPACITOR_0603  [CAPC1608X92N]
D4  MM3Z3V0B  ZENER_SOD-323  [SOD2514X100N]
D5  BAT54CW  A2K_SOT-323  [SOT65P210X110-3N]
D6  BAT54CW  A2K_SOT-323  [SOT65P210X110-3N]
D7  BAT54CW  A2K_SOT-323  [SOT65P210X110-3N]
D8  RB751S40  DIODE-SOD523  [SOD523]
D9  RB751S40  DIODE-SOD523  [SOD523]
J8  USB_A-VERTICAL  [USB-A-HU]
JP6  PINHD-2X4  [2X04]
R23  10K  RESISTOR_0603  [RESC1608X55N]
R24  10k  RESISTOR_0603  [RESC1608X55N]
R25  120R  RESISTOR_0603  [RESC1608X55N]
R26  10K  RESISTOR_0603  [RESC1608X55N]
RN17  51R  4R-NCAT16  [CAT16]
RN18  51R  4R-NCAT16  [CAT16]
RN19  49R9  2R-NEXBV4V  [EXBV4V]
U17  MK22DX256VLF5  MK22DX_VLF  [TQFP48]
Y2  TSX-3225 24MHz  XTAL_XRCGB  [XTAL_2.0X1.6]
Y3  32.768kHz  XTAL_9HT4  [9HT7]

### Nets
3V3_ARM: C62.2 C63.2 C66.2 D8.A D9.A JP6.7 R24.1 R26.1 U17.1(A:VDD) U17.5(B:VOUT33) U17.9(A:VDDA) U17.10(C:VREFH) U17.22(A:VDD)
!ARM_RESET: C68.2 JP6.8 R26.2 U17.26(D:!RESET)
!CFG_STAT: U17.31(F:PTB16) ; also sheet 5
!CONFIG: U17.32(F:PTB17) ; also sheet 5
!ETH_INT: U17.48(H:PTD7/TX0) ; also sheet 3,6
!EZP_CS: JP6.6 R24.2 U17.21(E:PTA4/!EZP_CS)
!I2C_IRQ: U17.29(F:PTB2) ; also sheet 2,6
!MENU/PWR: U17.47(H:PTD6/SPI0_PCS3/RX0) ; also sheet 1
!SPI_CS0: RN17.4 RN17.5 RN18.1 RN18.8 U17.41(H:PTD0/SPI0_PCS0) ; also sheet 3,6
!SPI_SEL1: RN18.3 RN18.6 U17.45(H:PTD4/SPI0_PCS1) ; also sheet 1,2
!SPI_SEL2: RN18.2 RN18.7 U17.35(G:PTC2/SPI0_PCS2/IS20_TX_FS) ; also sheet 1,2
+5V: D7.1(A1) ; also sheet 1
+5V/2: D7.2(A2) J8.VBUS(CN:VBUS) ; also sheet 1
CFG_DONE: U17.30(F:PTB3) ; also sheet 1,5
CONF_EN: RN18.4 RN18.5 U17.42(H:PTD1/SPI0_SCK) ; also sheet 3
GND: C61.1 C62.1 C63.1 C64.- C65.1 C66.1 C67.1 C68.1 D4.A J8.GND(CN:GND) J8.S@1(S:S1) J8.S@2(S:S2) J8.S@3(S:S3) J8.S@4(S:S4) JP6.3 R23.1 U17.2(A:VSS) U17.11(C:VREFL) U17.12(A:VSSA) U17.23(A:VSS) ; also sheet 1,2,3,5,6
I2C_SCL: U17.27(F:PTB0/I2C0_SCL) ; also sheet 2,6
I2C_SDA: U17.28(F:PTB1/I2C0_SDA) ; also sheet 2,6
KBD_CLK/RX2: D6.1(A1) U17.43(H:PTD2/SPI0_SOUT/RX2/I2C0_SCL) ; also sheet 2
KBD_DAT/TX2: D6.2(A2) U17.44(H:PTD3/SPI0_SIN/TX2/I2C0_SDA) ; also sheet 2
MS_CLK/RX1: D5.1(A1) U17.36(G:PTC3/SPI0_PCS1/RX1/IS20_TX_BLCK) ; also sheet 2
MS_DAT/TX1: D5.2(A2) U17.37(G:PTC4/SPI0_PCS0/TX1) ; also sheet 2
N$8: D4.K D5.3(K) D6.3(K)
N$52: U17.15(D:EXTAL32) Y3.1
N$53: U17.14(D:XTAL32) Y3.4
N$55: C67.2 D9.C R25.1 U17.16(D:VBAT)
N$63: U17.25(E:PTA19/XTAL0) Y2.3
N$64: C65.2 U17.13(C:VREF_OUT/CMP_IN5)
N$89: U17.24(E:PTA18/EXTAL0) Y2.1
N$95: RN19.4 U17.4(B:USB0_DM)
N$96: RN19.3 U17.3(B:USB0_DP)
N$100: C61.2 D7.3(K) D8.C U17.6(B:VREGIN)
N$121: C64.+ R25.2
PWR_EN: R23.2 U17.46(H:PTD5/SPI0_PCS2) ; also sheet 1
SPI_SCK: RN17.1 RN17.8 U17.38(G:PTC5/SPI0_SCK/I2S0_RXD0) ; also sheet 2,3,6
SPI_SEL3: U17.34(G:PTC1/SPI0_PCS3/I2S0_TXDO) ; also sheet 5
SPI_SEL4: U17.33(G:PTC0/SPI0_PCS4/ISS0_TXD1) ; also sheet 5
SPI_SIN: RN17.3 RN17.6 U17.40(G:PTC7/SPI0_SIN/I2S0_RX_FS) ; also sheet 2,3
SPI_SOUT: RN17.2 RN17.7 U17.39(G:PTC6/SPI0_SOUT/I2S0_RX_BCLK) ; also sheet 2,3,6
TCK/SWD_CLK/EZP_CLK: JP6.1 U17.17(E:PTA0/TCK/SWD_CLK/EZP_CLK)
TDI/EZP_DI/RXD0: JP6.2 U17.18(E:PTA1/TDI/RX0/EZP_DI)
TDO/EZP_DO/TXD0: JP6.4 U17.19(E:PTA2/TDO/TX0/EZP_DO)
TMS/SWD_DIO: JP6.5 U17.20(E:PTA3/TMS/SWD_DIO)
USB_D_N: J8.D-(CN:D-) RN19.1
USB_D_P: J8.D+(CN:D+) RN19.2
Unconnected: U17.7(C:ADC0_DM0) U17.8(C:ADC0_DP0)

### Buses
ALTERA_CONFIG
PERIPH_I/O
SPI

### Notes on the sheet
- protect LDO against
  back feeding 3.3V
  from DBG conn when 
  board not powered.
- ARM_3v3:
  +3.3V running
  +2.2V standby
- OTG acting as USB host
- Debug/Programming
  Connector
- Doc K20PB states K22 doesn't have any 5V tolerant I/O.
  Clamped signals to 3V zener as 3V3_ARM doesn't have much load.
  PWR_EN is active high because chip is not 5V tolerant
- This work is licensed under the Creative Commons
  Attribution-NonCommercial 4.0 International
  License. To view a copy of this license, visit
  http://creativecommons.org/licenses/by-nc/4.0/.
  
  Author: K. C. Lee
  "This work" = Schematic and hardware design
  
  PCB artwork: (C) 2014 Copyright All Reserved
- ARM Microcontroller

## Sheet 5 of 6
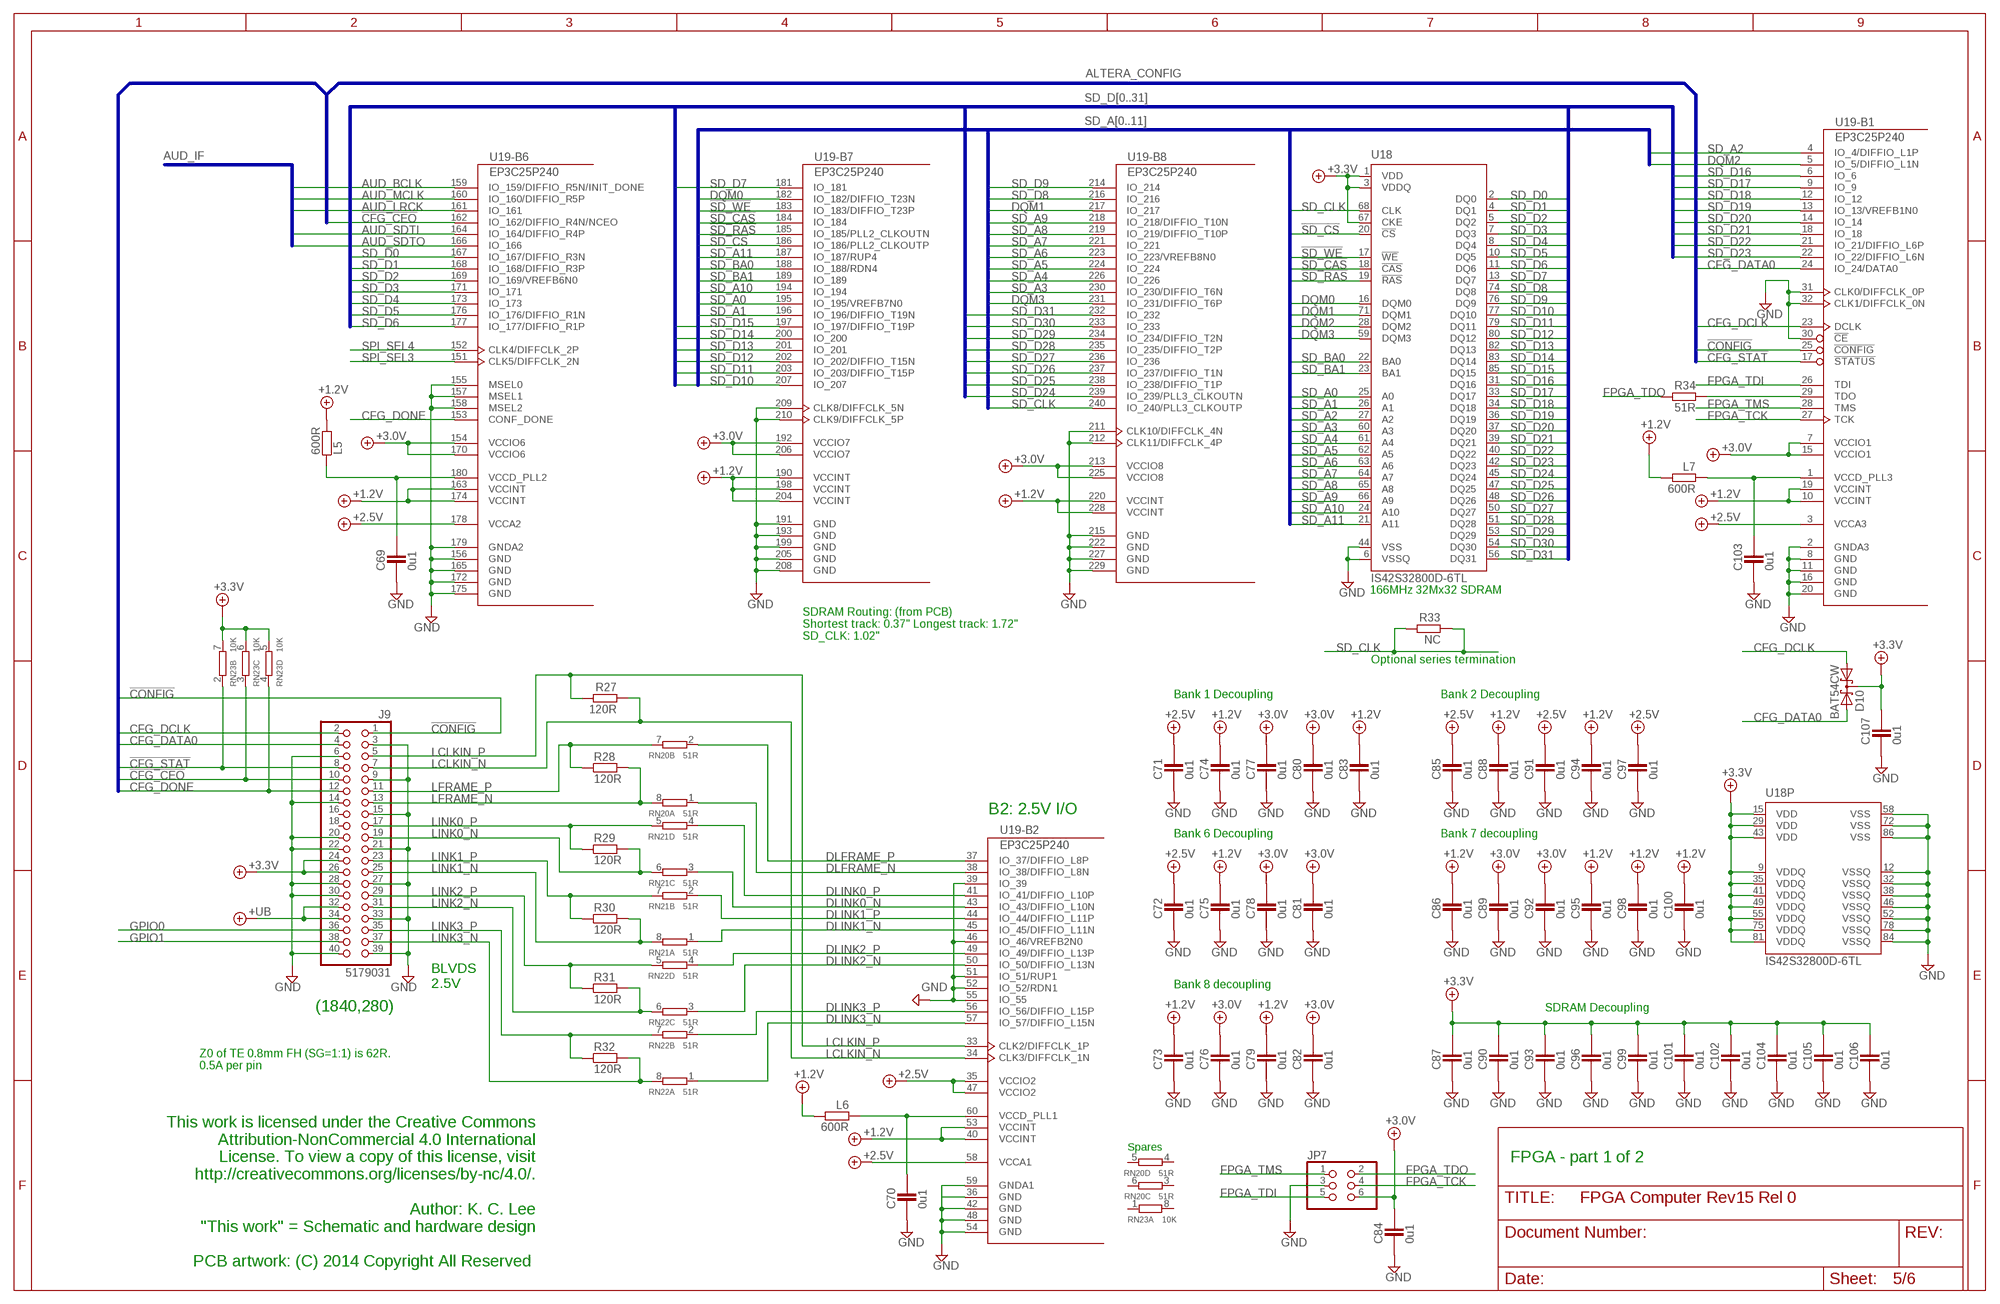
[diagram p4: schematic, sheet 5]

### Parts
C69  0u1  CAPACITOR_0402  [CAPC1005X60N]
C70  0u1  CAPACITOR_0603  [CAPC1608X92N]
C71  0u1  CAPACITOR_0402  [CAPC1005X60N]
C72  0u1  CAPACITOR_0402  [CAPC1005X60N]
C73  0u1  CAPACITOR_0402  [CAPC1005X60N]
C74  0u1  CAPACITOR_0402  [CAPC1005X60N]
C75  0u1  CAPACITOR_0402  [CAPC1005X60N]
C76  0u1  CAPACITOR_0402  [CAPC1005X60N]
C77  0u1  CAPACITOR_0402  [CAPC1005X60N]
C78  0u1  CAPACITOR_0402  [CAPC1005X60N]
C79  0u1  CAPACITOR_0402  [CAPC1005X60N]
C80  0u1  CAPACITOR_0402  [CAPC1005X60N]
C81  0u1  CAPACITOR_0402  [CAPC1005X60N]
C82  0u1  CAPACITOR_0402  [CAPC1005X60N]
C83  0u1  CAPACITOR_0402  [CAPC1005X60N]
C84  0u1  CAPACITOR_0603  [CAPC1608X92N]
C85  0u1  CAPACITOR_0603  [CAPC1608X92N]
C86  0u1  CAPACITOR_0402  [CAPC1005X60N]
C87  0u1  CAPACITOR_0402  [CAPC1005X60N]
C88  0u1  CAPACITOR_0402  [CAPC1005X60N]
C89  0u1  CAPACITOR_0402  [CAPC1005X60N]
C90  0u1  CAPACITOR_0603  [CAPC1608X92N]
C91  0u1  CAPACITOR_0402  [CAPC1005X60N]
C92  0u1  CAPACITOR_0402  [CAPC1005X60N]
C93  0u1  CAPACITOR_0603  [CAPC1608X92N]
C94  0u1  CAPACITOR_0402  [CAPC1005X60N]
C95  0u1  CAPACITOR_0402  [CAPC1005X60N]
C96  0u1  CAPACITOR_0603  [CAPC1608X92N]
C97  0u1  CAPACITOR_0402  [CAPC1005X60N]
C98  0u1  CAPACITOR_0402  [CAPC1005X60N]
C99  0u1  CAPACITOR_0603  [CAPC1608X92N]
C100  0u1  CAPACITOR_0402  [CAPC1005X60N]
C101  0u1  CAPACITOR_0402  [CAPC1005X60N]
C102  0u1  CAPACITOR_0603  [CAPC1608X92N]
C103  0u1  CAPACITOR_0402  [CAPC1005X60N]
C104  0u1  CAPACITOR_0603  [CAPC1608X92N]
C105  0u1  CAPACITOR_0402  [CAPC1005X60N]
C106  0u1  CAPACITOR_0402  [CAPC1005X60N]
C107  0u1  CAPACITOR_0603  [CAPC1608X92N]
D10  BAT54CW  A2K_SOT-323  [SOT65P210X110-3N]
J9  5179031  [TE-5179031-1]
JP7  PINHD-2X3_2.54-ROUND  [2X03-RND]
L5  600R  RESISTOR_0603  [RESC1608X55N]
L6  600R  RESISTOR_0603  [RESC1608X55N]
L7  600R  RESISTOR_0603  [RESC1608X55N]
R27  120R  RESISTOR_0402  [RESC1005X40AN]
R28  120R  RESISTOR_0402  [RESC1005X40AN]
R29  120R  RESISTOR_0402  [RESC1005X40AN]
R30  120R  RESISTOR_0402  [RESC1005X40AN]
R31  120R  RESISTOR_0402  [RESC1005X40AN]
R32  120R  RESISTOR_0402  [RESC1005X40AN]
R33  NC  RESISTOR_0402  [RESC1005X40AN]
R34  51R  RESISTOR_0603  [RESC1608X55N]
RN20  51R  4R-NCAT16  [CAT16]
RN21  51R  4R-NCAT16  [CAT16]
RN22  51R  4R-NCAT16  [CAT16]
RN23  10K  4R-NCAT16  [CAT16]
U18  IS42S32800D-6TL  MT48LC4M32B2  [TSOP86]
U19  EP3C25P240  [PQFP240]

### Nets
!CFG_CEO: J9.10 RN23.3 U19.162(-B6:IO_162/DIFFIO_R4N/NCEO)
!CFG_STAT: J9.8 RN23.2 U19.17(-B1:!STATUS) ; also sheet 4
!CONFIG: J9.1 U19.25(-B1:!CONFIG) ; also sheet 4
!SD_CAS: U18.18(!CAS) U19.184(-B7:IO_184)
!SD_CS: U18.20(!CS) U19.186(-B7:IO_186/PLL2_CLKOUTP)
!SD_RAS: U18.19(!RAS) U19.185(-B7:IO_185/PLL2_CLKOUTN)
!SD_WE: U18.17(!WE) U19.183(-B7:IO_183/DIFFIO_T23P)
+1.2V: C73.2 C74.2 C75.2 C79.2 C83.2 C86.2 C88.2 C94.2 C95.2 C98.2 C100.2 L5.2 L6.2 L7.2 U19.10(-B1:VCCINT) U19.19(-B1:VCCINT) U19.40(-B2:VCCINT) U19.53(-B2:VCCINT) U19.163(-B6:VCCINT) U19.174(-B6:VCCINT) U19.190(-B7:VCCINT) U19.198(-B7:VCCINT) U19.204(-B7:VCCINT) U19.220(-B8:VCCINT) U19.228(-B8:VCCINT) ; also sheet 1,6
+2.5V: C71.2 C72.2 C85.2 C91.2 C97.2 U19.3(-B1:VCCA3) U19.35(-B2:VCCIO2) U19.47(-B2:VCCIO2) U19.58(-B2:VCCA1) U19.178(-B6:VCCA2) ; also sheet 1,6
+3.0V: C76.2 C77.2 C78.2 C80.2 C81.2 C82.2 C84.2 C89.2 C92.2 JP7.6 U19.7(-B1:VCCIO1) U19.15(-B1:VCCIO1) U19.154(-B6:VCCIO6) U19.170(-B6:VCCIO6) U19.192(-B7:VCCIO7) U19.206(-B7:VCCIO7) U19.213(-B8:VCCIO8) U19.225(-B8:VCCIO8) ; also sheet 1,6
+3.3V: C87.2 C90.2 C93.2 C96.2 C99.2 C101.2 C102.2 C104.2 C105.2 C106.2 C107.2 D10.3(K) J9.24 J9.26 RN23.5 RN23.6 RN23.7 U18.1(VDD) U18.3(VDDQ) U18.9(VDDQ) U18.15(VDD) U18.29(VDD) U18.35(VDDQ) U18.41(VDDQ) U18.43(VDD) U18.49(VDDQ) U18.55(VDDQ) U18.67(CKE) U18.75(VDDQ) U18.81(VDDQ) ; also sheet 1,2,3
+UB: J9.32 J9.34 ; also sheet 1,2,6
AUD_BCLK: U19.159(-B6:IO_159/DIFFIO_R5N/INIT_DONE) ; also sheet 2
AUD_LRCK: U19.161(-B6:IO_161) ; also sheet 2
AUD_MCLK: U19.160(-B6:IO_160/DIFFIO_R5P) ; also sheet 2
AUD_SDTI: U19.164(-B6:IO_164/DIFFIO_R4P) ; also sheet 2
AUD_SDTO: U19.166(-B6:IO_166) ; also sheet 2
CFG_DATA0: D10.2(A2) J9.4 U19.24(-B1:IO_24/DATA0) ; also sheet 3
CFG_DCLK: D10.1(A1) J9.2 U19.23(-B1:DCLK) ; also sheet 3
CFG_DONE: J9.12 RN23.4 U19.153(-B6:CONF_DONE) ; also sheet 1,4
DLFRAME_N [diff2]: RN20.1 U19.38(-B2:IO_38/DIFFIO_L8N)
DLFRAME_P [diff2]: RN20.2 U19.37(-B2:IO_37/DIFFIO_L8P)
DLINK0_N [diff2]: RN21.3 U19.43(-B2:IO_43/DIFFIO_L10N)
DLINK0_P [diff2]: RN21.4 U19.41(-B2:IO_41/DIFFIO_L10P)
DLINK1_N [diff2]: RN21.1 U19.45(-B2:IO_45/DIFFIO_L11N)
DLINK1_P [diff2]: RN21.2 U19.44(-B2:IO_44/DIFFIO_L11P)
DLINK2_N [diff2]: RN22.3 U19.50(-B2:IO_50/DIFFIO_L13N)
DLINK2_P [diff2]: RN22.4 U19.49(-B2:IO_49/DIFFIO_L13P)
DLINK3_N [diff2]: RN22.1 U19.57(-B2:IO_57/DIFFIO_L15N)
DLINK3_P [diff2]: RN22.2 U19.56(-B2:IO_56/DIFFIO_L15P)
DQM0: U18.16(DQM0) U19.182(-B7:IO_182/DIFFIO_T23N)
DQM1: U18.71(DQM1) U19.217(-B8:IO_217)
DQM2: U18.28(DQM2) U19.5(-B1:IO_5/DIFFIO_L1N)
DQM3: U18.59(DQM3) U19.231(-B8:IO_231/DIFFIO_T6P)
FPGA_TCK: JP7.4 U19.27(-B1:TCK)
FPGA_TDI: JP7.5 U19.26(-B1:TDI)
FPGA_TDO: JP7.2 R34.2
FPGA_TMS: JP7.1 U19.28(-B1:TMS)
GND: C69.1 C70.1 C71.1 C72.1 C73.1 C74.1 C75.1 C76.1 C77.1 C78.1 C79.1 C80.1 C81.1 C82.1 C83.1 C84.1 C85.1 C86.1 C87.1 C88.1 C89.1 C90.1 C91.1 C92.1 C93.1 C94.1 C95.1 C96.1 C97.1 C98.1 C99.1 C100.1 C101.1 C102.1 C103.1 C104.1 C105.1 C106.1 C107.1 J9.3 J9.6 J9.9 J9.14 J9.15 J9.20 J9.21 J9.22 J9.27 J9.28 J9.30 J9.33 J9.39 J9.40 JP7.3 U18.6(VSSQ) U18.12(VSSQ) U18.32(VSSQ) U18.38(VSSQ) U18.44(VSS) U18.46(VSSQ) U18.52(VSSQ) U18.58(VSS) U18.72(VSS) U18.78(VSSQ) U18.84(VSSQ) U18.86(VSS) U19.2(-B1:GNDA3) U19.8(-B1:GND) U19.11(-B1:GND) U19.16(-B1:GND) U19.20(-B1:GND) U19.30(-B1:!CE) U19.31(-B1:CLK0/DIFFCLK_0P) U19.32(-B1:CLK1/DIFFCLK_0N) U19.36(-B2:GND) U19.39(-B2:IO_39) U19.42(-B2:GND) U19.46(-B2:IO_46/VREFB2N0) U19.48(-B2:GND) U19.51(-B2:IO_51/RUP1) U19.52(-B2:IO_52/RDN1) U19.54(-B2:GND) U19.55(-B2:IO_55) U19.59(-B2:GNDA1) U19.155(-B6:MSEL0) U19.156(-B6:GND) U19.157(-B6:MSEL1) U19.158(-B6:MSEL2) U19.165(-B6:GND) U19.172(-B6:GND) U19.175(-B6:GND) U19.179(-B6:GNDA2) U19.191(-B7:GND) U19.193(-B7:GND) U19.199(-B7:GND) U19.205(-B7:GND) U19.208(-B7:GND) U19.209(-B7:CLK8/DIFFCLK_5N) U19.210(-B7:CLK9/DIFFCLK_5P) U19.211(-B8:CLK10/DIFFCLK_4N) U19.212(-B8:CLK11/DIFFCLK_4P) U19.215(-B8:GND) U19.222(-B8:GND) U19.227(-B8:GND) U19.229(-B8:GND) ; also sheet 1,2,3,4,6
GPIO0: J9.36 ; also sheet 6
GPIO1: J9.38 ; also sheet 6
LCLKIN_N [diff2]: J9.7 R27.1 U19.34(-B2:CLK3/DIFFCLK_1N)
LCLKIN_P [diff2]: J9.5 R27.2 U19.33(-B2:CLK2/DIFFCLK_1P)
LFRAME_N [diff2]: J9.13 R28.2 RN20.8
LFRAME_P [diff2]: J9.11 R28.1 RN20.7
LINK0_N [diff2]: J9.19 R29.2 RN21.6
LINK0_P [diff2]: J9.17 R29.1 RN21.5
LINK1_N [diff2]: J9.25 R30.2 RN21.8
LINK1_P [diff2]: J9.23 R30.1 RN21.7
LINK2_N [diff2]: J9.31 R31.2 RN22.6
LINK2_P [diff2]: J9.29 R31.1 RN22.5
LINK3_N [diff2]: J9.37 R32.2 RN22.8
LINK3_P [diff2]: J9.35 R32.1 RN22.7
N$7: R34.1 U19.29(-B1:TDO)
N$40: C103.2 L7.1 U19.1(-B1:VCCD_PLL3)
N$41: C70.2 L6.1 U19.60(-B2:VCCD_PLL1)
N$42: C69.2 L5.1 U19.180(-B6:VCCD_PLL2)
SD_A0: U18.25(A0) U19.195(-B7:IO_195/VREFB7N0)
SD_A1: U18.26(A1) U19.196(-B7:IO_196/DIFFIO_T19N)
SD_A2: U18.27(A2) U19.4(-B1:IO_4/DIFFIO_L1P)
SD_A3: U18.60(A3) U19.230(-B8:IO_230/DIFFIO_T6N)
SD_A4: U18.61(A4) U19.226(-B8:IO_226)
SD_A5: U18.62(A5) U19.224(-B8:IO_224)
SD_A6: U18.63(A6) U19.223(-B8:IO_223/VREFB8N0)
SD_A7: U18.64(A7) U19.221(-B8:IO_221)
SD_A8: U18.65(A8) U19.219(-B8:IO_219/DIFFIO_T10P)
SD_A9: U18.66(A9) U19.218(-B8:IO_218/DIFFIO_T10N)
SD_A10: U18.24(A10) U19.194(-B7:IO_194)
SD_A11: U18.21(A11) U19.187(-B7:IO_187/RUP4)
SD_BA0: U18.22(BA0) U19.188(-B7:IO_188/RDN4)
SD_BA1: U18.23(BA1) U19.189(-B7:IO_189)
SD_CLK: R33.1 R33.2 U18.68(CLK) U19.240(-B8:IO_240/PLL3_CLKOUTP)
SD_D0: U18.2(DQ0) U19.167(-B6:IO_167/DIFFIO_R3N)
SD_D1: U18.4(DQ1) U19.168(-B6:IO_168/DIFFIO_R3P)
SD_D2: U18.5(DQ2) U19.169(-B6:IO_169/VREFB6N0)
SD_D3: U18.7(DQ3) U19.171(-B6:IO_171)
SD_D4: U18.8(DQ4) U19.173(-B6:IO_173)
SD_D5: U18.10(DQ5) U19.176(-B6:IO_176/DIFFIO_R1N)
SD_D6: U18.11(DQ6) U19.177(-B6:IO_177/DIFFIO_R1P)
SD_D7: U18.13(DQ7) U19.181(-B7:IO_181)
SD_D8: U18.74(DQ8) U19.216(-B8:IO_216)
SD_D9: U18.76(DQ9) U19.214(-B8:IO_214)
SD_D10: U18.77(DQ10) U19.207(-B7:IO_207)
SD_D11: U18.79(DQ11) U19.203(-B7:IO_203/DIFFIO_T15P)
SD_D12: U18.80(DQ12) U19.202(-B7:IO_202/DIFFIO_T15N)
SD_D13: U18.82(DQ13) U19.201(-B7:IO_201)
SD_D14: U18.83(DQ14) U19.200(-B7:IO_200)
SD_D15: U18.85(DQ15) U19.197(-B7:IO_197/DIFFIO_T19P)
SD_D16: U18.31(DQ16) U19.6(-B1:IO_6)
SD_D17: U18.33(DQ17) U19.9(-B1:IO_9)
SD_D18: U18.34(DQ18) U19.12(-B1:IO_12)
SD_D19: U18.36(DQ19) U19.13(-B1:IO_13/VREFB1N0)
SD_D20: U18.37(DQ20) U19.14(-B1:IO_14)
SD_D21: U18.39(DQ21) U19.18(-B1:IO_18)
SD_D22: U18.40(DQ22) U19.21(-B1:IO_21/DIFFIO_L6P)
SD_D23: U18.42(DQ23) U19.22(-B1:IO_22/DIFFIO_L6N)
SD_D24: U18.45(DQ24) U19.239(-B8:IO_239/PLL3_CLKOUTN)
SD_D25: U18.47(DQ25) U19.238(-B8:IO_238/DIFFIO_T1P)
SD_D26: U18.48(DQ26) U19.237(-B8:IO_237/DIFFIO_T1N)
SD_D27: U18.50(DQ27) U19.236(-B8:IO_236)
SD_D28: U18.51(DQ28) U19.235(-B8:IO_235/DIFFIO_T2P)
SD_D29: U18.53(DQ29) U19.234(-B8:IO_234/DIFFIO_T2N)
SD_D30: U18.54(DQ30) U19.233(-B8:IO_233)
SD_D31: U18.56(DQ31) U19.232(-B8:IO_232)
SPI_SEL3: U19.151(-B6:CLK5/DIFFCLK_2N) ; also sheet 4
SPI_SEL4: U19.152(-B6:CLK4/DIFFCLK_2P) ; also sheet 4
Unconnected: J9.16 J9.18 RN20.3 RN20.4 RN20.5 RN20.6 RN23.1 RN23.8

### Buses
SD_A[0..11]
SD_D[0..31]
ALTERA_CONFIG
AUD_IF

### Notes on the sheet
- 166MHz 32Mx32 SDRAM
- SDRAM Routing: (from PCB)
  Shortest track: 0.37" Longest track: 1.72"
  SD_CLK: 1.02"
- Optional series termination
- Bank 1 Decoupling | Bank 2 Decoupling
- B2: 2.5V I/O
- Bank 6 Decoupling | Bank 7 decoupling
- BLVDS
  2.5V
- Bank 8 decoupling
- (1840,280) | SDRAM Decoupling
- Z0 of TE 0.8mm FH (SG=1:1) is 62R.
  0.5A per pin
- Spares
- FPGA - part 1 of 2
- This work is licensed under the Creative Commons
  Attribution-NonCommercial 4.0 International
  License. To view a copy of this license, visit
  http://creativecommons.org/licenses/by-nc/4.0/.
  
  Author: K. C. Lee
  "This work" = Schematic and hardware design
  
  PCB artwork: (C) 2014 Copyright All Reserved

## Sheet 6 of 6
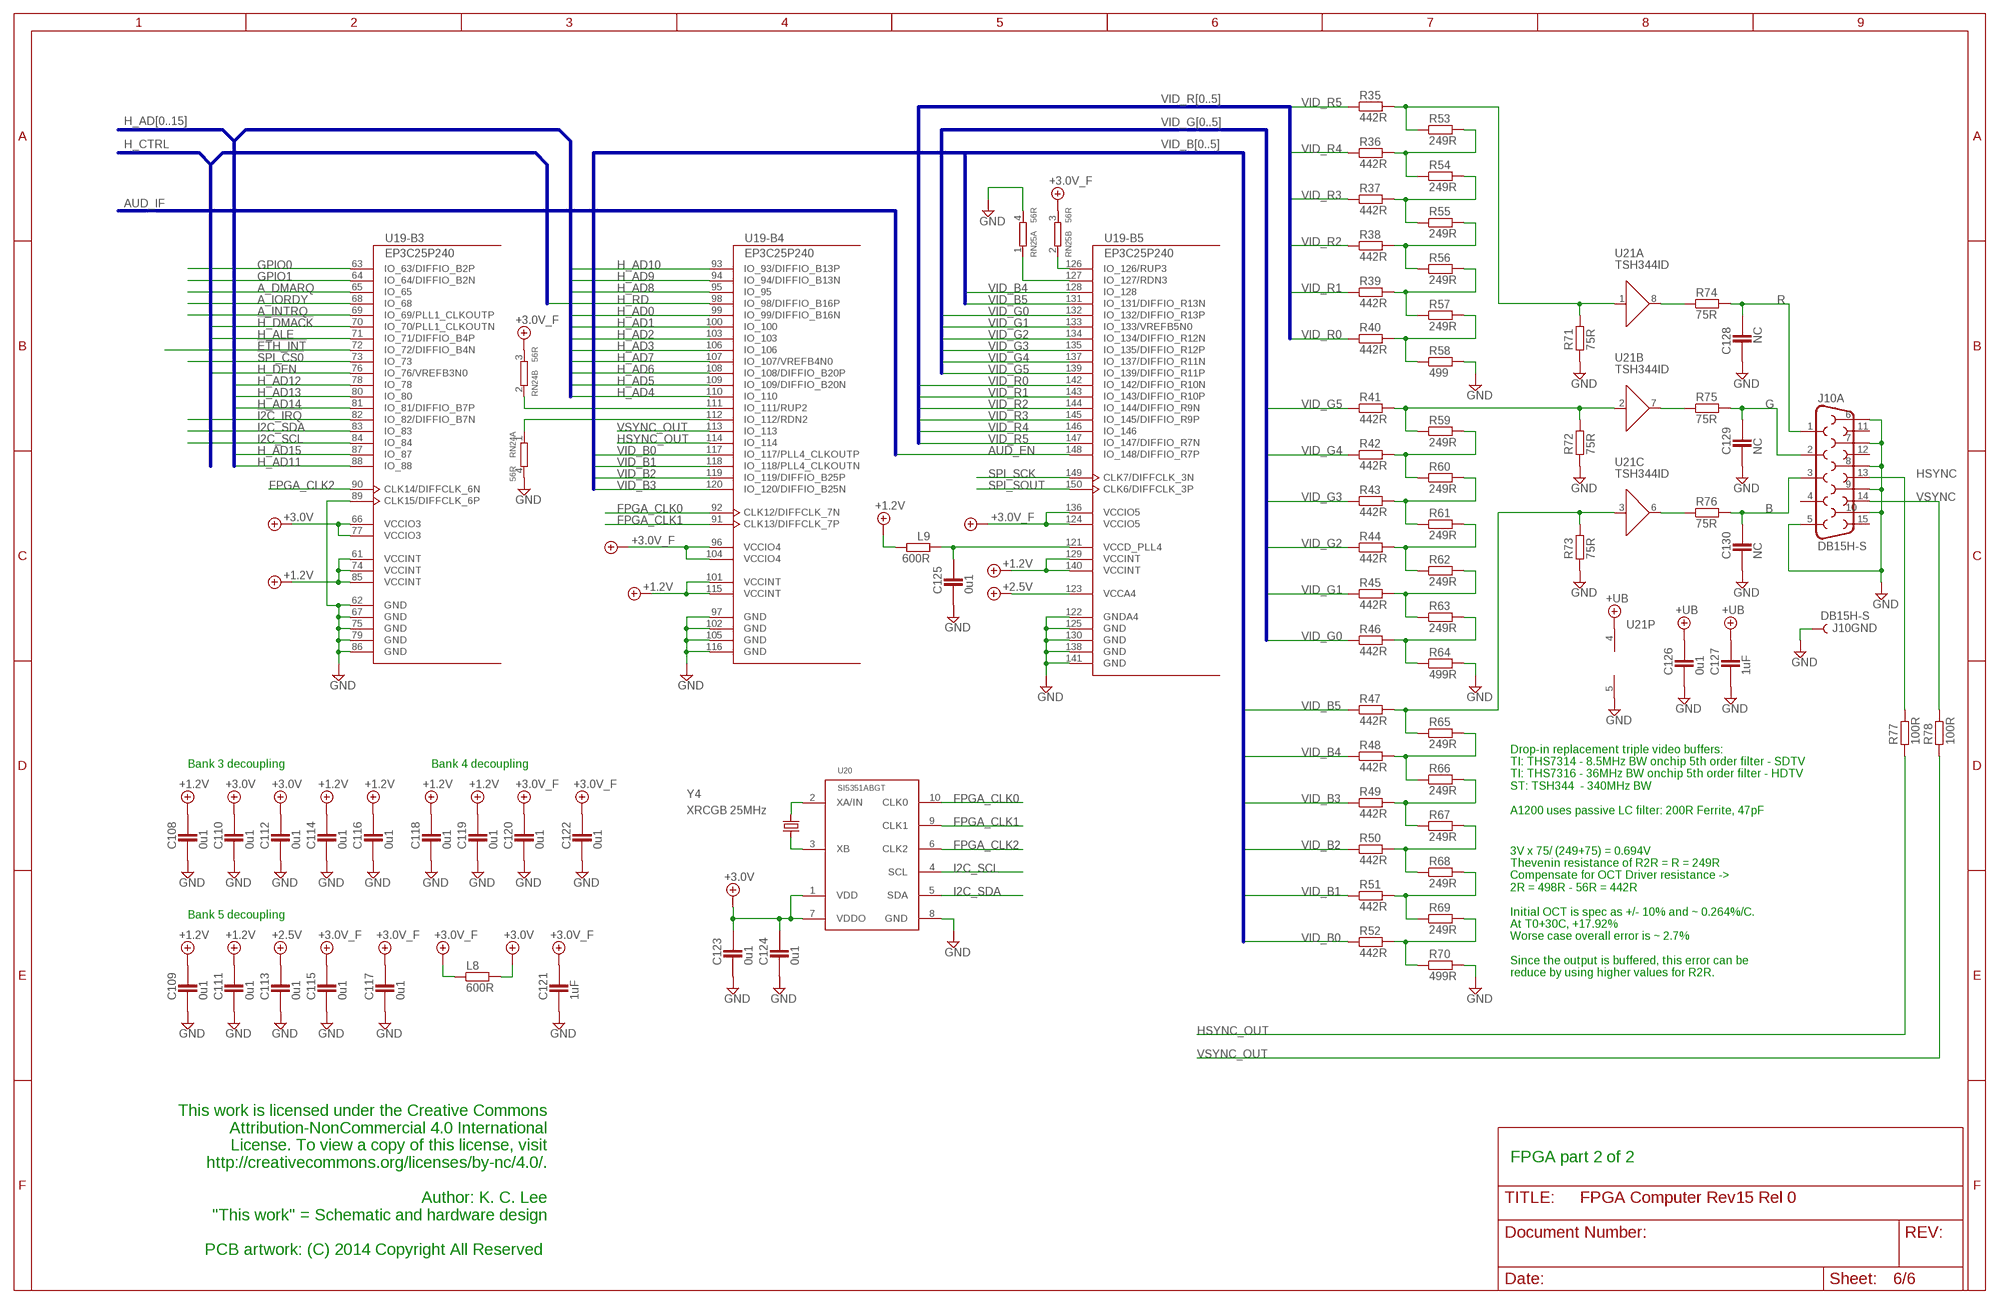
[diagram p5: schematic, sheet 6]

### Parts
C108  0u1  CAPACITOR_0402  [CAPC1005X60N]
C109  0u1  CAPACITOR_0402  [CAPC1005X60N]
C110  0u1  CAPACITOR_0402  [CAPC1005X60N]
C111  0u1  CAPACITOR_0402  [CAPC1005X60N]
C112  0u1  CAPACITOR_0402  [CAPC1005X60N]
C113  0u1  CAPACITOR_0402  [CAPC1005X60N]
C114  0u1  CAPACITOR_0402  [CAPC1005X60N]
C115  0u1  CAPACITOR_0402  [CAPC1005X60N]
C116  0u1  CAPACITOR_0402  [CAPC1005X60N]
C117  0u1  CAPACITOR_0402  [CAPC1005X60N]
C118  0u1  CAPACITOR_0402  [CAPC1005X60N]
C119  0u1  CAPACITOR_0402  [CAPC1005X60N]
C120  0u1  CAPACITOR_0402  [CAPC1005X60N]
C121  1uF  CAPACITOR_0603  [CAPC1608X92N]
C122  0u1  CAPACITOR_0402  [CAPC1005X60N]
C123  0u1  CAPACITOR_0603  [CAPC1608X92N]
C124  0u1  CAPACITOR_0402  [CAPC1005X60N]
C125  0u1  CAPACITOR_0402  [CAPC1005X60N]
C126  0u1  CAPACITOR_0603  [CAPC1608X92N]
C127  1uF  CAPACITOR_0603  [CAPC1608X92N]
C128  NC  CAPACITOR_0603  [CAPC1608X92N]
C129  NC  CAPACITOR_0603  [CAPC1608X92N]
C130  NC  CAPACITOR_0603  [CAPC1608X92N]
J10  DB15H-S  [DB15HS]
L8  600R  RESISTOR_0603  [RESC1608X55N]
L9  600R  RESISTOR_0603  [RESC1608X55N]
R35  442R  RESISTOR_0402  [RESC1005X40AN]
R36  442R  RESISTOR_0402  [RESC1005X40AN]
R37  442R  RESISTOR_0402  [RESC1005X40AN]
R38  442R  RESISTOR_0402  [RESC1005X40AN]
R39  442R  RESISTOR_0402  [RESC1005X40AN]
R40  442R  RESISTOR_0402  [RESC1005X40AN]
R41  442R  RESISTOR_0402  [RESC1005X40AN]
R42  442R  RESISTOR_0402  [RESC1005X40AN]
R43  442R  RESISTOR_0402  [RESC1005X40AN]
R44  442R  RESISTOR_0402  [RESC1005X40AN]
R45  442R  RESISTOR_0402  [RESC1005X40AN]
R46  442R  RESISTOR_0402  [RESC1005X40AN]
R47  442R  RESISTOR_0402  [RESC1005X40AN]
R48  442R  RESISTOR_0402  [RESC1005X40AN]
R49  442R  RESISTOR_0402  [RESC1005X40AN]
R50  442R  RESISTOR_0402  [RESC1005X40AN]
R51  442R  RESISTOR_0402  [RESC1005X40AN]
R52  442R  RESISTOR_0402  [RESC1005X40AN]
R53  249R  RESISTOR_0402  [RESC1005X40AN]
R54  249R  RESISTOR_0402  [RESC1005X40AN]
R55  249R  RESISTOR_0402  [RESC1005X40AN]
R56  249R  RESISTOR_0402  [RESC1005X40AN]
R57  249R  RESISTOR_0402  [RESC1005X40AN]
R58  499  RESISTOR_0402  [RESC1005X40AN]
R59  249R  RESISTOR_0402  [RESC1005X40AN]
R60  249R  RESISTOR_0402  [RESC1005X40AN]
R61  249R  RESISTOR_0402  [RESC1005X40AN]
R62  249R  RESISTOR_0402  [RESC1005X40AN]
R63  249R  RESISTOR_0402  [RESC1005X40AN]
R64  499R  RESISTOR_0402  [RESC1005X40AN]
R65  249R  RESISTOR_0402  [RESC1005X40AN]
R66  249R  RESISTOR_0402  [RESC1005X40AN]
R67  249R  RESISTOR_0402  [RESC1005X40AN]
R68  249R  RESISTOR_0402  [RESC1005X40AN]
R69  249R  RESISTOR_0402  [RESC1005X40AN]
R70  499R  RESISTOR_0402  [RESC1005X40AN]
R71  75R  RESISTOR_0603  [RESC1608X55N]
R72  75R  RESISTOR_0603  [RESC1608X55N]
R73  75R  RESISTOR_0603  [RESC1608X55N]
R74  75R  RESISTOR_0603  [RESC1608X55N]
R75  75R  RESISTOR_0603  [RESC1608X55N]
R76  75R  RESISTOR_0603  [RESC1608X55N]
R77  100R  RESISTOR_0603  [RESC1608X55N]
R78  100R  RESISTOR_0603  [RESC1608X55N]
RN24  56R  2R-NEXBV4V  [EXBV4V]
RN25  56R  2R-NEXBV4V  [EXBV4V]
U20  SI5351ABGT  [MSOP-10]
U21  TSH344ID  [SO-8]
Y4  XRCGB 25MHz  XTAL_XRCGB  [XTAL_2.0X1.6]

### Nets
!ETH_INT: U19.72(-B3:IO_72/DIFFIO_B4N) ; also sheet 3,4
!H_DMACK: U19.70(-B3:IO_70/PLL1_CLKOUTN) ; also sheet 3
!I2C_IRQ: U19.82(-B3:IO_82/DIFFIO_B7N) ; also sheet 2,4
!SPI_CS0: U19.73(-B3:IO_73) ; also sheet 3,4
+1.2V: C108.2 C109.2 C111.2 C114.2 C116.2 C118.2 C119.2 L9.2 U19.61(-B3:VCCINT) U19.74(-B3:VCCINT) U19.85(-B3:VCCINT) U19.101(-B4:VCCINT) U19.115(-B4:VCCINT) U19.129(-B5:VCCINT) U19.140(-B5:VCCINT) ; also sheet 1,5
+2.5V: C113.2 U19.123(-B5:VCCA4) ; also sheet 1,5
+3.0V: C110.2 C112.2 C123.2 C124.2 L8.2 U19.66(-B3:VCCIO3) U19.77(-B3:VCCIO3) U20.1(VDD) U20.7(VDDO) ; also sheet 1,5
+3.0V_F: C115.2 C117.2 C120.2 C121.2 C122.2 L8.1 RN24.3 RN25.3 U19.96(-B4:VCCIO4) U19.104(-B4:VCCIO4) U19.124(-B5:VCCIO5) U19.136(-B5:VCCIO5)
+UB: C126.2 C127.2 U21.4(P:V+) ; also sheet 1,2,5
A_DMARQ: U19.65(-B3:IO_65) ; also sheet 3
A_INTRQ: U19.69(-B3:IO_69/PLL1_CLKOUTP) ; also sheet 3
A_IORDY: U19.68(-B3:IO_68) ; also sheet 3
AUD_EN: U19.148(-B5:IO_148/DIFFIO_R7P) ; also sheet 2
B: C130.2 J10.3 R76.2
FPGA_CLK0: U19.92(-B4:CLK12/DIFFCLK_7N) U20.10(CLK0)
FPGA_CLK1: U19.91(-B4:CLK13/DIFFCLK_7P) U20.9(CLK1)
FPGA_CLK2: U19.90(-B3:CLK14/DIFFCLK_6N) U20.6(CLK2)
G: C129.2 J10.2 R75.2
GND: C108.1 C109.1 C110.1 C111.1 C112.1 C113.1 C114.1 C115.1 C116.1 C117.1 C118.1 C119.1 C120.1 C121.1 C122.1 C123.1 C124.1 C125.1 C126.1 C127.1 C128.2 C129.1 C130.1 J10.5 J10.6 J10.7 J10.8 J10.9 J10.10 J10.G1(GND:B) J10.G2(GND:B) R58.2 R64.2 R70.2 R71.1 R72.1 R73.1 RN24.4 RN25.4 U19.62(-B3:GND) U19.67(-B3:GND) U19.75(-B3:GND) U19.79(-B3:GND) U19.86(-B3:GND) U19.89(-B3:CLK15/DIFFCLK_6P) U19.97(-B4:GND) U19.102(-B4:GND) U19.105(-B4:GND) U19.116(-B4:GND) U19.122(-B5:GNDA4) U19.125(-B5:GND) U19.130(-B5:GND) U19.138(-B5:GND) U19.141(-B5:GND) U20.8(GND) U21.5(P:V-) ; also sheet 1,2,3,4,5
GPIO0: U19.63(-B3:IO_63/DIFFIO_B2P) ; also sheet 5
GPIO1: U19.64(-B3:IO_64/DIFFIO_B2N) ; also sheet 5
H_AD0: U19.99(-B4:IO_99/DIFFIO_B16N) ; also sheet 3
H_AD1: U19.100(-B4:IO_100) ; also sheet 3
H_AD2: U19.103(-B4:IO_103) ; also sheet 3
H_AD3: U19.106(-B4:IO_106) ; also sheet 3
H_AD4: U19.110(-B4:IO_110) ; also sheet 3
H_AD5: U19.109(-B4:IO_109/DIFFIO_B20N) ; also sheet 3
H_AD6: U19.108(-B4:IO_108/DIFFIO_B20P) ; also sheet 3
H_AD7: U19.107(-B4:IO_107/VREFB4N0) ; also sheet 3
H_AD8: U19.95(-B4:IO_95) ; also sheet 3
H_AD9: U19.94(-B4:IO_94/DIFFIO_B13N) ; also sheet 3
H_AD10: U19.93(-B4:IO_93/DIFFIO_B13P) ; also sheet 3
H_AD11: U19.88(-B3:IO_88) ; also sheet 3
H_AD12: U19.78(-B3:IO_78) ; also sheet 3
H_AD13: U19.80(-B3:IO_80) ; also sheet 3
H_AD14: U19.81(-B3:IO_81/DIFFIO_B7P) ; also sheet 3
H_AD15: U19.87(-B3:IO_87) ; also sheet 3
H_ALE: U19.71(-B3:IO_71/DIFFIO_B4P) ; also sheet 3
H_DEN: U19.76(-B3:IO_76/VREFB3N0) ; also sheet 3
H_RD: U19.98(-B4:IO_98/DIFFIO_B16P) ; also sheet 3
HSYNC: J10.13 R77.2
HSYNC_OUT: R77.1 U19.114(-B4:IO_114)
I2C_SCL: U19.84(-B3:IO_84) U20.4(SCL) ; also sheet 2,4
I2C_SDA: U19.83(-B3:IO_83) U20.5(SDA) ; also sheet 2,4
N$2: U20.3(XB) Y4.1
N$6: R40.2 R57.2 R58.1
N$21: R39.2 R56.2 R57.1
N$23: R35.2 R53.1 R71.2 U21.1(A:IN)
N$26: R47.2 R65.1 R73.2 U21.3(C:IN)
N$27: R41.2 R59.1 R72.2 U21.2(B:IN)
N$33: C125.2 L9.1 U19.121(-B5:VCCD_PLL4)
N$34: R42.2 R59.2 R60.1
N$35: R43.2 R60.2 R61.1
N$36: R36.2 R53.2 R54.1
N$37: R37.2 R54.2 R55.1
N$38: R38.2 R55.2 R56.1
N$39: R44.2 R61.2 R62.1
N$43: RN25.2 U19.126(-B5:IO_126/RUP3)
N$44: RN25.1 U19.127(-B5:IO_127/RDN3)
N$45: R48.2 R65.2 R66.1
N$46: R49.2 R66.2 R67.1
N$47: R50.2 R67.2 R68.1
N$48: RN24.2 U19.111(-B4:IO_111/RUP2)
N$49: RN24.1 U19.112(-B4:IO_112/RDN2)
N$50: R51.2 R68.2 R69.1
N$57: R46.2 R63.2 R64.1
N$58: R52.2 R69.2 R70.1
N$59: R45.2 R62.2 R63.1
N$62: R76.1 U21.6(C:OUT)
N$68: U20.2(XA/IN) Y4.3
N$92: R75.1 U21.7(B:OUT)
N$94: R74.1 U21.8(A:OUT)
R: C128.1 J10.1 R74.2
SPI_SCK: U19.149(-B5:CLK7/DIFFCLK_3N) ; also sheet 2,3,4
SPI_SOUT: U19.150(-B5:CLK6/DIFFCLK_3P) ; also sheet 2,3,4
VID_B0: R52.1 U19.117(-B4:IO_117/PLL4_CLKOUTP)
VID_B1: R51.1 U19.118(-B4:IO_118/PLL4_CLKOUTN)
VID_B2: R50.1 U19.119(-B4:IO_119/DIFFIO_B25P)
VID_B3: R49.1 U19.120(-B4:IO_120/DIFFIO_B25N)
VID_B4: R48.1 U19.128(-B5:IO_128)
VID_B5: R47.1 U19.131(-B5:IO_131/DIFFIO_R13N)
VID_G0: R46.1 U19.132(-B5:IO_132/DIFFIO_R13P)
VID_G1: R45.1 U19.133(-B5:IO_133/VREFB5N0)
VID_G2: R44.1 U19.134(-B5:IO_134/DIFFIO_R12N)
VID_G3: R43.1 U19.135(-B5:IO_135/DIFFIO_R12P)
VID_G4: R42.1 U19.137(-B5:IO_137/DIFFIO_R11N)
VID_G5: R41.1 U19.139(-B5:IO_139/DIFFIO_R11P)
VID_R0: R40.1 U19.142(-B5:IO_142/DIFFIO_R10N)
VID_R1: R39.1 U19.143(-B5:IO_143/DIFFIO_R10P)
VID_R2: R38.1 U19.144(-B5:IO_144/DIFFIO_R9N)
VID_R3: R37.1 U19.145(-B5:IO_145/DIFFIO_R9P)
VID_R4: R36.1 U19.146(-B5:IO_146)
VID_R5: R35.1 U19.147(-B5:IO_147/DIFFIO_R7N)
VSYNC: J10.14 R78.2
VSYNC_OUT: R78.1 U19.113(-B4:IO_113)
Unconnected: J10.4 J10.11 J10.12 J10.15

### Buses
VID_R[0..5]
VID_G[0..5]
VID_B[0..5]
AUD_IF
H_CTRL
H_AD[0..15]

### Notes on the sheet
- Bank 3 decoupling | Bank 4 decoupling
- Drop-in replacement triple video buffers: 
  TI: THS7314 - 8.5MHz BW onchip 5th order filter - SDTV
  TI: THS7316 - 36MHz BW onchip 5th order filter - HDTV
  ST: TSH344  - 340MHz BW
  
  A1200 uses passive LC filter: 200R Ferrite, 47pF
- Bank 5 decoupling
- 3V x 75/ (249+75) = 0.694V
  Thevenin resistance of R2R = R = 249R
  Compensate for OCT Driver resistance -> 
  2R = 498R - 56R = 442R
  
  Initial OCT is spec as +/- 10% and ~ 0.264%/C.
  At T0+30C, +17.92%  
  Worse case overall error is ~ 2.7%
  
  Since the output is buffered, this error can be
  reduce by using higher values for R2R.
- FPGA part 2 of 2
- This work is licensed under the Creative Commons
  Attribution-NonCommercial 4.0 International
  License. To view a copy of this license, visit
  http://creativecommons.org/licenses/by-nc/4.0/.
  
  Author: K. C. Lee
  "This work" = Schematic and hardware design
  
  PCB artwork: (C) 2014 Copyright All Reserved

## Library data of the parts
C1-C5 C7-C14 C16-C18 C20-C24 C26 C27 C30 C32-C34 C37-C48 C50-C63 C65-C130 = ipc-7351-capacitor:CAPACITOR_
C6 C15 C25 C31 = ipc-7351-capacitor:POLARISED_
C19 = Misc Passives:CAP_POL: Capacitor Polarized
C28 C29 = rcl:CPOL-EU: POLARIZED CAPACITOR, European symbol
C35 C36 = Misc Passives:C-PR-1
C64 = Misc Passives:PAS: 3.8mm dia x 1.1mm Seiko XH311HUIV07E, Taiyo Yuden PAS311HR-VG1
D1 = Misc opto:DUAL-LED: LEDs
D2 = Misc opto:1204-SIDE-DUAL
D3 D8 D9 = diode:DIODE-: DIODE
D4 = ipc-7351-diode:ZENER_
D5-D7 D10 = Misc Passives:A2K_
H1-H4 = FPGA board Rev10:MOUNT-PAD-ROUND: MOUNTING PAD, round
J1 = Misc Conn:DCJ0202: DC POWER JACK Source: DCJ0202.pdf Pin = CUI Inc. PJ-102A with formed pins
J2 J3 = Misc Conn:PINHD-2X5: PIN HEADER
J4 = Misc Conn:MINI_DIN_6
J5 = Misc Conn:TE-1932739
J6 = Misc Conn:STX-4235: Kycon: stx-4235-3/3-N (Mouser) CUI: SJD-3510-33 [Discontinued] (Digikey)
J7 = Misc Conn:HR911105A
J8 = Misc Conn:USB_A: FCI 73725-0110BLF Vertical USB A
J9 = Misc Conn:5179031: TE Plug assembly FH 0.8mm - 40 pos.
J10 = Misc Conn:DB15H-S: DB15 / VGA right angle through-hole female connector.
JP1 = Misc Conn:SCREW-TERM: Screw Terminal:
JP2 JP4 JP7 = Misc Conn:PINHD-2X3: PIN HEADER
JP3 = pinhead-1:PINHD-1X6: PIN HEADER
JP5 = Misc Conn:PINHD-2X22: PIN HEADER
JP6 = Misc Conn:PINHD-2X4: PIN HEADER
L1 L4-L9 R1-R78 = ipc-7351-resistor:RESISTOR_
L2 L3 = Misc Inductors:NRS4018
PTC1 PTC2 = microbuilder:PTC: PTC (Resettable Fuse); DIGIKEY_PART#: F2152CT-ND
PTC3 PTC4 = microbuilder:PTC: PTC (Resettable Fuse)
Q1 = ipc-7351-transistor:MOSFET-NCH_
RN1-RN7 RN10-RN18 RN20-RN23 = Misc Passives:4R-N: Array Chip Resistor Source: RS Component / Phycomp; OC_FARNELL: unknown; OC_NEWARK: unknown
RN8 RN9 RN19 RN24 RN25 = Misc Passives:2R-N: Array Chip Resistor Source: Panasonic; OC_FARNELL: unknown; OC_NEWARK: unknown
S1 = Misc Passives:MOM_SW-RT: OMRON SWITCH
TP1-TP9 = testpad:TPSQ: Test pad
U1 = Misc Logic:74LVC1G11
U2 = 74xx-little-us:74*1G04: INVERTER Gate
U3 = Misc Power:AP25X1: Diodes Inc. 2.5A Current-limited power switch
U4 = Misc Power:TCM809XX: Power supply supervisor.
U5 = Misc Power:PAM2306D
U6 U7 = Misc Power:MCP1700
U8 U12 = Misc Power:LDO-5
U9 = Misc Analog:AK4556VT
U10 = Misc Peripherals:XRA1201: Exar I2C 8-bit expander
U11 = Misc Analog:TPA6139A2: TI Headphone amplifier - Audio path
U13 = Misc Memory:25*: Serial memory, SPI bus; DIGIKEY_PART#: 1274-1045-ND; MF: MICROCHIP; MPN: 25LC080/SN; OC_FARNELL: 1137302; OC_NEWARK: 96K4092
U14 = Misc PLD:XC9572VQ64
U15 = Misc Peripherals:ENC624J600: Ethernet 10/100
U16 = Misc Logic:74LVC3G17
U17 = Misc Processor:MK22DX_V: Freescale Cortex M4 in 48 pin package: MK22DX128VLF5, MK22DX256VLF5
U18 = memory-micron (fixed):MT48LC4M32B2: SYNCHRONOUS DRAM 1 Meg x 32 x 4 banks Source: http://www.datasheetcatalog.org/datasheet/micron/MT48LC4M32B2.pdf; MPN: MT48LC4M32B2P-6:G; OC_FARNELL: 1216286; OC_NEWARK: 97K6124
U19 = Misc PLD:EP3C25
U20 = Misc Clock:SI5351ABGT
U21 = Misc Analog:TSH344
Y1-Y4 = Misc Clock:XTAL_: kHz RANGE CRYSTAL UNIT

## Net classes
0 signals: width 0.203 mm, clearance 0.152 mm
2 diff: width 0.305 mm, clearance 0.203 mm
3 diff2: width 0.203 mm, clearance 0.205 mm to class 0, clearance 0.205 mm to class 1, clearance 0.205 mm to class 2, clearance 0.203 mm

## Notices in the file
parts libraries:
microbuilder: This work is placed in the public domain, and may be freely used for commercial and non-commercial work with the following conditions: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
